(* Logix 5000 Rung export; software revision 16.04 *)

MODULES
   Local : vendor None type None code None
   PDPMV1_FLEX : vendor None type None code None
END_MODULES

TYPE PDPMV1_Status :   // Status data from the MVI56-PDPMV1 module
STRUCT
   Pattern : SINT[12];   // Module indentification code
   Input_Size : INT;   // Configured PROFIBUS input data size
   Output_Size : INT;   // Configured PROFIBUS output data size
   Reserved1 : INT;   // Not Used
   Reserved2 : INT;   // Not Used
   Reserved3 : INT;   // Not Used
   Input_Swap : SINT;   // Configured input swap byte option (1=swap bytes, 0= no swap)
   Output_Swap : SINT;   // Configured output swap byte option (1=swap bytes, 0= no swap)
   Module_Major_Ver : SINT;   // Module major firmware version
   Module_Minor_Ver : SINT;   // Module minor firmware version
   Fieldbus : PDPMV1_Fieldbus;   // PROFIBUS network status information
   Control : PDPMV1_StatusControl;   // Module information
   Profibus_CRC32 : DINT;   // CRC value related to the PROFIBUS configuration that was downloaded to the module
   Module_CRC32 : DINT;   // CRC value related to the module configuration that was downloaded to the module
   Module : PDPMV1_Module;   // General module status to monitor data, mailbox and alarm exchange between the processor and the module
   Backplane : PDPMV1_backplane;   // Backplane status information
   Other : PDPMV1_other_status;   // General mailbox and cfg error information
END_STRUCT
END_TYPE

TYPE PDPMV1_GetSlaveConfig_Out :   // GetSlaveConfig mailbox request
STRUCT
   SlaveAddress : INT;   // Destination of slave (1-125)
END_STRUCT
END_TYPE

TYPE PDPMV1_MSGUtil :   // Data structure for each MSG type that monitors if the message execution is sucessfull
STRUCT
   DNCounter : COUNTER;   // Incremented once the MSG done bit is set (PRE=100000)
   ERCounter : COUNTER;   // Incremented once the MSG ER bit is set (PRE=100000)
   LastError : INT;   // Last Error Code received
   Pending : BOOL;   // Indicates that the message is executing and the processor is waiting for its conclusion (DN or ER)
END_STRUCT
END_TYPE

TYPE PDPMV1_GetSlaveConfig_In :   // GetSlaveConfig mailbox response from a specific slave
STRUCT
   ByteCount : INT;   // Byte count data block
   SlaveAddress : INT;   // Destination of slave (1-125)
   ErrorCode : INT[1];   // If other than 0, refer to user manual for code information
   ReturnCode : INT;   // If other than 0, refer to user manual for code information
   FaultInformation : INT;   // If other than 0, refer to user manual for code information
   Identifier : SINT[245];   // Configuration from a specific connected PROFIBUS slave
END_STRUCT
END_TYPE

TYPE PDPMV1_StopSlave_Out :   // Mailbox request
STRUCT
   SlaveNumber : SINT[126];   // Slave number designation (1-125)
END_STRUCT
END_TYPE

TYPE PDPMV1_Control :   // This data structure contains the command bits to request mailbox, retrieve status and request reboot from the module
STRUCT
   AcyclicRead : BOOL;   // Request the module to send acyclic read message to slave
   AcyclicWrite : BOOL;   // Request the module to send acyclic write message to slave
   GetLiveList : BOOL;   // Request the Live List information from the module
   GetSlaveConfig : BOOL;   // Request configuration information from a slave
   GetSlaveDiagnostics : BOOL;   // Requests slave diagnostics from a slave
   GetStatus : BOOL;   // Request for status information from the module
   Reboot : BOOL;   // Request the module reboot
   SetClearMode : BOOL;   // Set the module to clear mode (outputs are disabled)
   SetOperateMode : BOOL;   // Set the module to operate mode (module only communicates through PROFIBUS)
   SetStopMode : BOOL;   // Set the module to stop mode (PROFIBUS communication is interrupted in stop mode)
   SetSlaveAddress : BOOL;   // Change the slave's PROFIBUS address (only if slave supports this feature)
   SetSlaveMode : BOOL;   // Set the slave mode to Synch, Freeze, Unsynch, Unfreeze
   StartSlaves : BOOL;   // Restarts PROFIBUS communication with one or more slaves after a "StopSlave" mailbox
   StopSlaves : BOOL;   // Stop PROFIBUS communication with one or more slaves
END_STRUCT
END_TYPE

TYPE PDPMV1_StartSlaves :   // StartSlaves mailbox allows the processor to restart communication to slaves that were previoulsy interrupted by StopSlaves
STRUCT
   Out : PDPMV1_StartSlaves_Out;   // Mailbox Request
   In : PDPMV1_StartSlaves_In;   // Mailbox Response
END_STRUCT
END_TYPE

TYPE PDPMV1_GetSlaveDiagnostics_In :   // GetSlaveDiagnostics mailbox response
STRUCT
   RequestType : SINT;   // Type of request. 0 to use module memory RAM or 1 for live PROFIBUS network.
   SlaveAddress : SINT;   // Destination of slave (1-125)
   ExtendedFaultInfo : INT;   // If other than 0, refer to user manual for code information
   FaultInformation : INT;   // If other than 0, refer to user manual for code information
   StationStatus1_2 : INT;   // Status of station types 1 and 2
   StationStatus3_4 : INT;   // Status of station types 3 and 4
   IdentNumber : INT;   // Unique ID assigned by the PROFIBUS User Organization
   ExtendedDiagnosticData : INT[200];   // Slave user-specific data. Refer to actual slave documentation for info
END_STRUCT
END_TYPE

TYPE PDPMV1_Alarm :   // DPV1 alarm data received by the module
STRUCT
   ByteCount : INT;   // Byte count data block
   SlotNumber : SINT;   // Used in the slave to address the desired data block. Range 0-254
   SlaveAddress : SINT;   // Destination of slave (1-125)
   AlarmSpecAck : SINT;   // Additional alarm information
   SeqNumber : SINT;   // Unique ID number of the alarm. Range 0-31.
   ExtDiag : SINT;   // Extended Diagnostic Flag (FFh - flag set and 00h - flag cleared).
   AlarmType : SINT;   // Identifies alarm type. Range is from 1 to 6, 32 to 126.
   FaultInformation : INT;   // If other than 0, refer to user manual for code information
   Data : SINT[500];   // Returned data [1...n] array with additional manf. spec alarm info.
END_STRUCT
END_TYPE

TYPE PDPMV1_Connection_Output :   // Connection input to be associated to the module
STRUCT
   Data : INT[69];   // Backplane output connection type - change the array size for your application
END_STRUCT
END_TYPE

TYPE PDPMV1_AcyclicRead_In :   // DPV1 acyclic read mailbox response
STRUCT
   ByteCount : INT;   // Byte count data block
   SlotNumber : SINT;   // Used in the slave to address the desired data block.
   SlaveAddress : SINT;   // Destination of slave (1-125)
   Length : SINT;   // Specifies the number of bytes of the data block to read
   Index : SINT;   // Index block
   ErrorDecode : SINT;   // If other than 0, refer to user manual for code information
   ErrorCode2 : SINT;   // If other than 0, refer to user manual for code information
   ErrorCode1 : SINT;   // If other than 0, refer to user manual for code information
   ExtendedFaultInfo : INT;   // If other than 0, refer to user manual for code information
   FaultInformation : INT;   // If other than 0, refer to user manual for code information
   Data : SINT[200];   // Returned data [1...n] array
END_STRUCT
END_TYPE

TYPE PDPMV1_PROFIBUS_IOSize :   // This type is used to store the module configuration input and output parameters
STRUCT
   InputDataSize : INT;   // Total PROFIBUS input word count configured through PCB.
   OutputDataSize : INT;   // Total PROFIBUS output word count configured through PCB.
END_STRUCT
END_TYPE

TYPE PDPMV1_AcyclicRead_Out :   // DPV1 acyclic read mailbox request
STRUCT
   SlotNumber : SINT;   // Used in the slave to address the desired data block.
   SlaveAddress : SINT;   // Destination of slave (1-125)
   DataSize : INT;   // Object data size
   Length : SINT;   // Specifies the number of bytes of the data block to read
   Index : SINT;   // Index block
END_STRUCT
END_TYPE

TYPE PDPMV1_UTIL :   // Contains registers used for ladder usage (these should not be updated by user application)
STRUCT
   CurrentAlarm : INT;   // New alarm index received from the module.
   CurrentMailbox : INT;   // New current mailbox index received from the module
   LastRead : INT;   // Last read block index received from the module
   ReadBlockIDOffset : INT;   // Read Block ID offset in Read Block
   LastWrite : INT;   // Last write block index received from the module
   BlockIndex : INT;   // Block index of each copy of PROFIBUS input and output blocks
   ReadBlockCount : INT;   // Number of read blocks transferred by the module to the processor
   WriteBlockCount : INT;   // Number of write blocks transferred by the processor to the module
   ReadBlockSize : INT;   // Input total size configured through RSLogix and reported by the module
   WriteBlockSize : INT;   // Output total size configured through RSLogix and reported by the module
   OutputWordsPerWriteBlock : INT;   // Word count reserved for PROFIBUS output data. All write blocks will use this amount except possibly last block.
   InputWordsPerReadBlock : INT;   // Word count reserved for PROFIBUS input data. All read blocks will use this amount except possibly last block.
   InputBytesPerReadBlock : INT;   // Byte count reserved for PROFIBUS input data. All read blocks will use this amount except possibly last block.
   OutputWordsInLastWriteBlock : INT;   // Word count with PROFIBUS output data in the last write block.
   InputWordsInLastReadBlock : INT;   // Word count with PROFIBUS input data in the last read block.
   InputBytesInLastReadBlock : INT;   // Byte count with PROFIBUS intput data in the last read block.
   MailboxInBuffer : INT[144];   // Mailbox response buffer received from the module. The content will be handled according to its mailbox ID
   MailboxOutBuffer : INT[144];   // Output mailbox buffer
   AlarmBuffer : INT[144];   // Buffer that stores the received alarm information
   StatusBuffer : INT[76];   // Buffer that stores the received status information
   MailboxIDOutLowByte : INT;   // Mailbox ID incremented for every mailbox request. Occupies the low byte of mailbox ID word register
   MailboxIDOut : INT;   // Final MailboxID for request mailbox. Corresponds to MailboxIDOutLowByte at low byte and "-20480" at high byte
   MailboxIDIn : INT;   // Received mailbox ID from the module - will match the corresponding request mailbox ID
   ByteSwapUtil : INT;   // Used for byte swap logic
   TempInt : INT;   // Used for integer formatting
   MSG : PDPMV1_MSGUtilTotal;   // Control Registers for MSG operation
END_STRUCT
END_TYPE

TYPE PDPMV1_AcyclicRead :   // DPV1 acyclic read mailbox data structure
STRUCT
   Out : PDPMV1_AcyclicRead_Out;   // mailbox request
   In : PDPMV1_AcyclicRead_In;   // mailbox response
END_STRUCT
END_TYPE

TYPE PDPMV1_SetSlaveMode :   // SetSlaveMode mailbox that allows the processor to change the slave mode to interrupt input or output data update
STRUCT
   Out : PDPMV1_SetSlaveMode_Out;   // Mailbox Request
   In : PDPMV1_SetSlaveMode_In;   // Mailbox Response
END_STRUCT
END_TYPE

TYPE PDPMV1_GetSlaveDiagnostics_Out :   // GetSlaveDiagnostics mailbox request
STRUCT
   RequestType : SINT;   // Type of request. 0 to use module memory RAM or 1 for live PROFIBUS network.
   SlaveAddress : SINT;   // Destination of slave (1-125)
END_STRUCT
END_TYPE

TYPE PDPMV1_Module :   // Status data
STRUCT
   Mod_scan_count : INT;   // Incremented every module scan loop
   Mod_output_update : INT;   // Incremented at every output scan
   Mod_input_update : INT;   // Incremented at every input scan
   Mod_out_MB : INT;   // Incremented at every output mailbox processing
   Mod_in_MB : INT;   // Incremented at every intput mailbox processing
   Mod_alarm_ind : INT;   // Incremented at every alarm indication
   Mod_alarm_con : INT;   // Incremented at every alarm confirmation
   Mod_acyclic_read : INT;   // Reserved
   Mod_acyclic_write : INT;   // Reserved
END_STRUCT
END_TYPE

TYPE PDPMV1_GetSlaveConfig :   // GetSlaveConfig mailobox to retrieve configuration data from specific PROFIBUS slaves
STRUCT
   Out : PDPMV1_GetSlaveConfig_Out;   // mailbox request
   In : PDPMV1_GetSlaveConfig_In;   // mailbox response
END_STRUCT
END_TYPE

TYPE PDPMV1_Connection_Input :   // Connection input to be associated to the module
STRUCT
   Data : INT[72];   // Backplane input connection type - change the array size for your application
END_STRUCT
END_TYPE

TYPE PDPMV1_GetSlaveDiagnostics :   // GetSlaveDiagnostics mailbox to retrieve diagnostic information from specific PROFIBUS slaves
STRUCT
   Out : PDPMV1_GetSlaveDiagnostics_Out;   // Mailbox request
   In : PDPMV1_GetSlaveDiagnostics_In;   // Mailbox response
END_STRUCT
END_TYPE

TYPE PDPMV1_StopSlave_In :   // Mailbox response
STRUCT
   AdditionalFaultinfo : INT;   // If other than 0, refer to user manual for code information
   FaultInformation : INT;   // If other than 0, refer to user manual for code information
   SlaveNumber : SINT[126];   // Slave number designation (1-125)
END_STRUCT
END_TYPE

TYPE PDPMV1_StartSlaves_In :   // Mailbox Response
STRUCT
   AdditionalFaultInfo : INT;   // If other than 0, refer to user manual for code information
   FaultInformation : INT;   // If other than 0, refer to user manual for code information
   SlaveNumber : SINT[126];   // Slave number designation (1-125)
END_STRUCT
END_TYPE

TYPE PDPMV1_GetLiveList :   // GetLiveList mailbox to retrieve the live list information from PROFIBUS network, informing the slaves that are communicating
STRUCT
   ReturnCode : SINT;   // Returned code about the nodes on the network
   FaultInfo : SINT;   // If other than 0, refer to user manual for code information
   Station : SINT[127];   // Station type contents.
END_STRUCT
END_TYPE

TYPE PDPMV1_ModuleDefinition :   // Main module definition
STRUCT
   PROFIBUSData : PDPMV1_Data;   // PROFIBUS data transferred between the processor and the PROFIBUS network
   Config : PDPMV1_Configuration;   // Module configuration information (backplane block sizes and PROFIBUS data sizes)
   Command : PDPMV1_Control;   // Command bits for special tasks and mailbox requests
   Mailbox : PDPMV1_Mailbox;   // Mailbox tags for optional applications
   Status : PDPMV1_Status;   // Module status information
   Util : PDPMV1_UTIL;   // Internal tags used for ladder logic processing. User applications should not overwrite any Util tags
END_STRUCT
END_TYPE

TYPE PDPMV1_Mailbox :   // Stores all mailbox request and response registers
STRUCT
   AcyclicRead : PDPMV1_AcyclicRead;   // This encapsulates a DPV1 Class 1 acyclic read request.
   AcyclicWrite : PDPMV1_AcyclicWrite;   // This encapsulates a DPV1 Class 1 acyclic write request.
   Alarm : PDPMV1_Alarm;   // This indicates to the application that a DPV1 slave has transferred an Alarm message to the master.
   GetLiveList : PDPMV1_GetLiveList;   // This command returns 127 bytes of information about the nodes on the network.
   GetSlaveConfig : PDPMV1_GetSlaveConfig;   // This command reads the actual configuration (identifier bytes) of a specified slave.
   GetSlaveDiagnostics : PDPMV1_GetSlaveDiagnostics;   // This command reads diagnostic data from a specified slave.
   SetSlaveAddress : PDPMV1_SetSlaveAddress;   // This command makes it possible to set the node address of a specified slave, if the slave supports this feature.
   SetSlaveMode : PDPMV1_SetSlaveMode;   // This control command is transmitted as multicast commands.
   StartSlaves : PDPMV1_StartSlaves;   // This mailbox message starts a selection of slaves that was previously removed from the processing cycle by means of the mailbox
   StopSlaves : PDPMV1_StopSlave;   // This mailbox message stops a selection of slaves from the processing cycle.
END_STRUCT
END_TYPE

TYPE PDPMV1_SetSlaveMode_In :   // Mailbox response
STRUCT
   GroupSelect : SINT;   // Range 01h to FFh (Bit Coded). This parameter determines which group to address. Refer to the user manual for examples
   SlaveAddress : SINT;   // Range 1 to 125; 127 (Multicast address).
   ControlCommand : PDPMV1_ControlCommand;   // This parameter specifies the command to send (Unsync/Sync and Unfreeze/Freeze).
   ExtendedFaultInfo : INT;   // If other than 0, refer to user manual for code information
   FaultInformation : INT;   // If other than 0, refer to user manual for code information
END_STRUCT
END_TYPE

TYPE PDPMV1_AcyclicWrite_In :   // DPV1 acyclic write mailbox response
STRUCT
   ByteCount : INT;   // Byte count data block
   SlotNumber : SINT;   // Used in the slave to address the desired data block.
   SlaveAddress : SINT;   // Destination of slave (1-125)
   Length : SINT;   // Specifies the number of bytes of the data block to read
   Index : SINT;   // Index block
   ErrorDecode : SINT;   // If other than 0, refer to user manual for code information
   ErrorCode2 : SINT;   // If other than 0, refer to user manual for code information
   ErrorCode1 : SINT;   // If other than 0, refer to user manual for code information
   ExtendedFaultInfo : INT;   // If other than 0, refer to user manual for code information
   FaultInformation : INT;   // If other than 0, refer to user manual for code information
   Data : SINT[200];   // Returned data [1...n] array
END_STRUCT
END_TYPE

TYPE PDPMV1_SetSlaveAddress_In :   // Mailbox response
STRUCT
   ByteCount : INT;   // Byte count data block
   NewSlaveAddress : SINT;   // Range 1 to 125, specifies the new address of the slave.
   CurrentSlaveAddress : SINT;   // Range 1 to 125, specifies the current address of the slave.
   SlaveIdentNumber : INT;   // Ident number for the slave, which address should be altered.
   No_add_Chg : INT;   // This parameter specifies whether it is allowed to change the slave address again
   ErrorCode1_2 : INT;   // If other than 0, refer to user manual for code information
   ErrorCode3_4 : INT;   // If other than 0, refer to user manual for code information
   ReturnCode : INT;   // If other than 0, refer to user manual for code information
   FaultInformation : INT;   // If other than 0, refer to user manual for code information
   MessageDataByte : SINT[400];   // Message data byte array for user-specific data
END_STRUCT
END_TYPE

TYPE PDPMV1_StatusControl :   // Module general information
STRUCT
   serial_number : SINT[4];   // Module serial number
   version_MSB : SINT;   // Module version number (most significant byte)
   version_LSB : SINT;   // Module version number (least significant byte)
   mod_status_MSB : SINT;   // Module status (most significant byte)
   mod_status_LSB : SINT;   // Module status (least significant byte)
END_STRUCT
END_TYPE

TYPE PDPMV1_ControlCommand :   // Option bits for SetSlaveMode mailbox
STRUCT
   Reserved1 : BOOL;   // Reserved
   Reserved2 : BOOL;   // Reserved
   Unfreeze_Input : BOOL;   // Freeze mode is concluded when initiated
   Freeze_Input : BOOL;   // Causes the addressed slave to assume freeze mode.
   Unsynchronize_Output : BOOL;   // Unsynchronized output data
   Synchronize_Output : BOOL;   // Synchronized output data
   Reserved3 : BOOL[32];   // Reserved
END_STRUCT
END_TYPE

TYPE PDPMV1_SetSlaveMode_Out :   // Mailbox Request
STRUCT
   GroupSelect : SINT;   // Range 01h to FFh (Bit Coded). This parameter determines which group to address. Refer to the user manual for examples
   SlaveAddress : SINT;   // Range 1 to 125; 127 (Multicast address).
   ControlCommand : PDPMV1_ControlCommand;   // This parameter specifies the command to send (Unsync/Sync and Unfreeze/Freeze).
END_STRUCT
END_TYPE

TYPE PDPMV1_Backplane_IOSize :   // This type is used to store the module configuration input and output parameters
STRUCT
   ReadBlockSize : INT;   // Total read (input) block size in words set for 1756-MODULE profile through RSLogix (from 12 through 250 words)
   WriteBlockSize : INT;   // Total write (output) block size in words set for 1756-MODULE profile through RSLogix (from 5 through 248 words)
END_STRUCT
END_TYPE

TYPE PDPMV1_StartSlaves_Out :   // Mailbox Request
STRUCT
   SlaveNumber : SINT[126];   // Slave number designation (1-125)
END_STRUCT
END_TYPE

TYPE PDPMV1_SetSlaveAddress :   // SetSlaveAddress mailbox that allows the module to dynamically change a PRIDUBUS address (only for slaves that supports it)
STRUCT
   Out : PDPMV1_SetSlaveAddress_Out;   // Mailbox request
   In : PDPMV1_SetSlaveAddress_In;   // Mailbox response
END_STRUCT
END_TYPE

TYPE PDPMV1_MSGUtilTotal :   // Stores all registers that are used to monitor MSG execution.
STRUCT
   MailboxRequest : PDPMV1_MSGUtil;   // Registers for monitoring of request mailbox MSG instructions
   MailboxResponse : PDPMV1_MSGUtil;   // Registers for monitoring of response mailbox MSG instructions
   GetStatus : PDPMV1_MSGUtil;   // Registers for monitoring of get status MSG instructions
   GetAlarm : PDPMV1_MSGUtil;   // Registers for monitoring of rget alarm MSG instructions
END_STRUCT
END_TYPE

TYPE PDPMV1_AcyclicWrite :   // DPV1 acyclic write mailbox data structure
STRUCT
   Out : PDPMV1_AcyclicWrite_Out;   // Mailbox request
   In : PDPMV1_AcyclicWrite_In;   // Mailbox response
END_STRUCT
END_TYPE

TYPE PDPMV1_StopSlave :   // StopSlaves mailbox allows the processor to interrupt communication to specific PROFIBUS slaves
STRUCT
   Out : PDPMV1_StopSlave_Out;   // Mailbox Request
   In : PDPMV1_StopSlave_In;   // Mailbox Response
END_STRUCT
END_TYPE

TYPE PDPMV1_SetSlaveAddress_Out :   // Mailbox request
STRUCT
   ByteCount : INT;   // Byte count data block
   NewSlaveAddress : SINT;   // Range 1 to 125, specifies the new address of the slave.
   CurrentSlaveAddress : SINT;   // Range 1 to 125, specifies the current address of the slave.
   SlaveIdentNumber : INT;   // Ident number for the slave, which address should be altered.
   No_add_Chg : INT;   // This parameter specifies whether it is allowed to change the slave address again
   MessageDataByte : SINT[400];   // Message data byte array for user-specific data
END_STRUCT
END_TYPE

TYPE PDPMV1_Data :   // PROFIBUS data transferred between the processor and and the PROFIBUS slaves
STRUCT
   Input : SINT[1536];   // Input PROFIBUS data (from module to processor)
   Output : SINT[1536];   // Output PROFIBUS data (from processor to module)
END_STRUCT
END_TYPE

TYPE PDPMV1_backplane :   // Stores variables used by sample ladder logic for handshaking purposes.
STRUCT
   Read : INT;   // Backplane read statistics
   Write : INT;   // Backplane write statistics
   Error : INT;   // Backplane error statistics
END_STRUCT
END_TYPE

TYPE PDPMV1_other_status :
STRUCT
   Cfg_file_error : INT;   // Bit0 = PDPMV1.CFG, Bit 1 = WATTCP.CFG, Bit 2 = PDPMV1.DDB, Bit3=PDPMV1.XML
   Reserved0 : INT;   // Not Used
   Reserved1 : INT;   // Not Used
   Reserved2 : INT;   // Not Used
   Reserved3 : INT;   // Not Used
   Reserved4 : INT;   // Not Used
   Reserved5 : INT;   // Not Used
   Reserved6 : INT;   // Not Used
   Reserved7 : INT;   // Not Used
   Reserved8 : INT;   // Not Used
   Reserved9 : INT;   // Not Used
   Reserved10 : INT;   // Not Used
   Reserved11 : INT;   // Not Used
   Reserved12 : INT;   // Not Used
   In_MB_queue : INT;   // Number of messages in the input mailbox queue
   Out_MB_queue : INT;   // Number of messages in the output mailbox queue
   Alarm_MB_queue : INT;   // Number of messages in the alarm mailbox queue
END_STRUCT
END_TYPE

TYPE PDPMV1_Fieldbus :
STRUCT
   FB_Slave_Cfg_List : SINT[16];   // Bitmap structure containing PROFIBUS slave configuration (bit x = 1 means slave x is configured)
   FB_Slave_Data_xfer : SINT[16];   // Bitmap structure containing PROFIBUS slave data exchange status (bit x = 1 means slave x is transferring data to the module)
   FB_Slave_Diag : SINT[16];   // Bitmap structure containing PROFIBUS slave diagnostic info (bit x = 1 means slave x is reporting diagnostics)
   FB_Pad_Byte : SINT;   // Reserved
   FB_op_state : SINT;   // Operation state ( 00 = offline, 40 = stop, 80 = clear, C0= operate)
   FB_ident_MSB : SINT;   // Master identification code (most significant byte)
   FB_ident_LSB : SINT;   // Master identification code (least significant byte)
END_STRUCT
END_TYPE

TYPE PDPMV1_Configuration :   // Stores current module configuration read from the module. The module cannot be configured from ladder.
STRUCT
   Backplane : PDPMV1_Backplane_IOSize;   // This tag will contain the input and output backplane block sizes configured by the user for the module through RSLogix
   PROFIBUS : PDPMV1_PROFIBUS_IOSize;   // This tag will contain the input and output PROFIBUS sizes configured by the user for the module through PCB
   PROFIBUS_CRC : DINT;   // Contains the CRC value (32-bits) associated to the module configuration file
   Module_CRC : DINT;   // Contains the CRC value (32-bits) associated to the PROFIBUSconfiguration file
END_STRUCT
END_TYPE

TYPE PDPMV1_AcyclicWrite_Out :   // DPV1 acyclic write mailbox request
STRUCT
   SlotNumber : SINT;   // Used in the slave to address the desired data block.
   SlaveAddress : SINT;   // Destination of slave (1-125)
   DataSize : INT;   // Object data size
   Length : SINT;   // Specifies the number of bytes of the data block to read
   Index : SINT;   // Index block
   Data : SINT[200];   // Data that should be written [1...n]
END_STRUCT
END_TYPE

ADD_ON_INSTRUCTION AOI56PDPMV1_FLEX   (* revision 1.5, vendor ProSoft Technology Inc., ExecutePrescan *)
// Add-On for the MVI56-PDPMV1 (Flexible I/O) module.
// Revision note:
// v1.5 - Commands that require messaging can now be accessed more than once after power up or mode change.
VAR_IN_OUT
   Connection_Input : PDPMV1_Connection_Input; {required}
   Connection_Output : PDPMV1_Connection_Output; {required}
   MVI56PDPMV1 : PDPMV1_ModuleDefinition; {required}
   AcyclicRead_MSG : MESSAGE; {required}   // Message tag for Acyclic Read mailbox request
   AcyclicWrite_MSG : MESSAGE; {required}   // Message tag for Acyclic Write mailbox request
   GetAlarm_MSG : MESSAGE; {required}   // Message tag for Get Alarm mailbox request
   GetMailbox_MSG : MESSAGE; {required}   // Message tag to retrieve mailbox response
   GetStatus_MSG : MESSAGE; {required}   // Message tag to retrieve module status
   GetLiveList_MSG : MESSAGE; {required}   // Message tag for Get Live List mailbox request
   GetSlaveCfg_MSG : MESSAGE; {required}   // Message tag for Get Slave Configuration mailbox request
   GetSlaveDiagnostics_MSG : MESSAGE; {required}   // Message tag for Get Slave Diagnostics mailbox request
   SetClearMode_MSG : MESSAGE; {required}   // Message tag for Set Clear Mode mailbox request
   SetOperateMode_MSG : MESSAGE; {required}   // Message tag for Set Operate Mode mailbox request
   SetSlaveAddress_MSG : MESSAGE; {required}   // Message tag for Set Slave Address mailbox request
   SetSlaveMode_MSG : MESSAGE; {required}   // Message tag for Set Slave Mode mailbox
   SetStopMode_MSG : MESSAGE; {required}   // Message tag for Set Stop mode mailbox request
   StartSlaves_MSG : MESSAGE; {required}   // Message tag for Start Slaves mailbox request
   StopSlaves_MSG : MESSAGE; {required}   // Message tag for Stop Slaves mailbox request
END_VAR
VAR
   MJFAULTS : DINT[12];
END_VAR

ROUTINE Logic   (* ladder *)
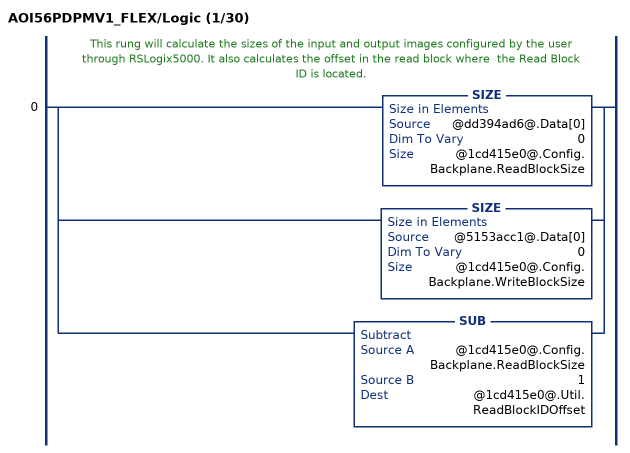
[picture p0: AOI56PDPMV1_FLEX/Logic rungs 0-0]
   // This rung will calculate the sizes of the input and output images configured by the user through RSLogix5000. It also calculates the offset in the read block where  the Read Block ID is located.
   0: [SIZE(@dd394ad6@.Data[0],0,@1cd415e0@.Config.Backplane.ReadBlockSize) ,SIZE(@5153acc1@.Data[0],0,@1cd415e0@.Config.Backplane.WriteBlockSize) ,SUB(@1cd415e0@.Config.Backplane.ReadBlockSize,1,@1cd415e0@.Util.ReadBlockIDOffset) ];
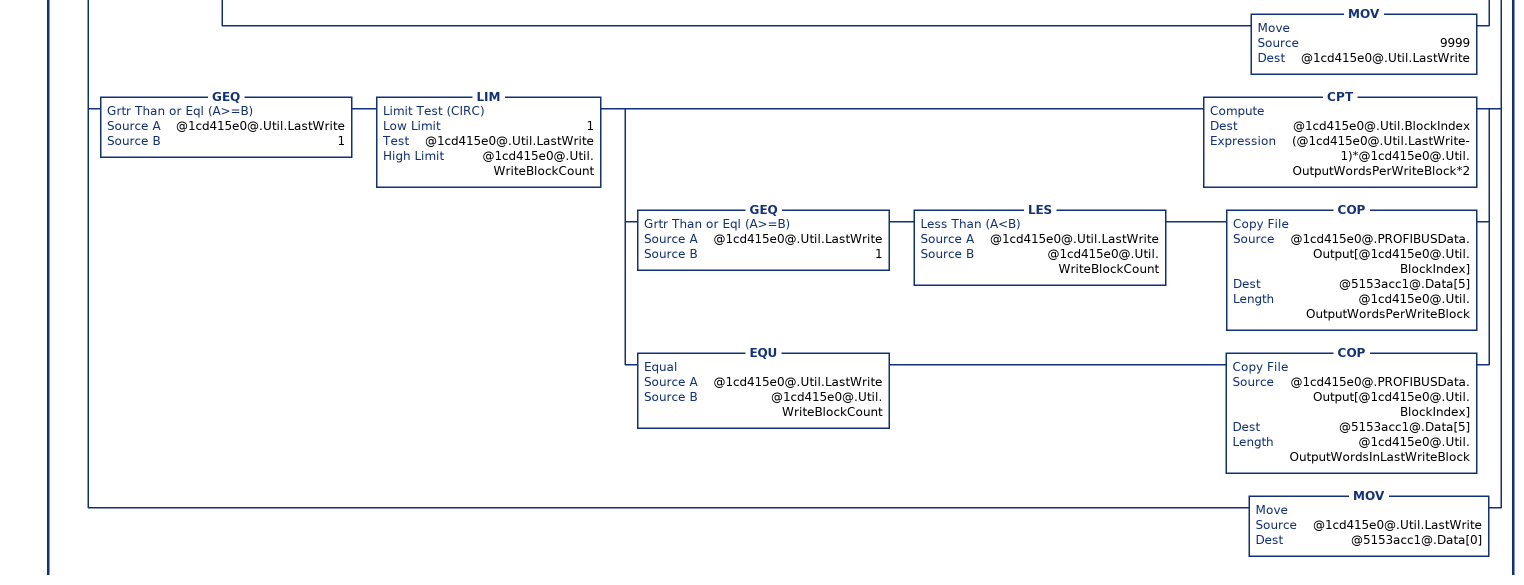
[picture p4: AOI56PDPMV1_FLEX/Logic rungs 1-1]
   // The new received read block ID is copied to the MVI56PDPMV1.Util.LastRead controller tag to guarantee that this logic will be performed one time only for each new bloc.
   1: NEQ(@dd394ad6@.Data[@1cd415e0@.Util.ReadBlockIDOffset],@1cd415e0@.Util.LastRead)[MOV(@dd394ad6@.Data[@1cd415e0@.Util.ReadBlockIDOffset],@1cd415e0@.Util.LastRead) ,EQU(@dd394ad6@.Data[0],9990) EQU(@1cd415e0@.Util.LastRead,9990) [MOV(@dd394ad6@.Data[1],@1cd415e0@.Util.ReadBlockSize) ,MOV(@dd394ad6@.Data[2],@1cd415e0@.Util.WriteBlockSize) ,MOV(@dd394ad6@.Data[3],@1cd415e0@.Config.PROFIBUS.InputDataSize) ,MOV(@dd394ad6@.Data[4],@1cd415e0@.Config.PROFIBUS.OutputDataSize) ,MOV(@dd394ad6@.Data[5],@1cd415e0@.Util.ReadBlockCount) ,MOV(@dd394ad6@.Data[6],@1cd415e0@.Util.WriteBlockCount) ,MOV(@dd394ad6@.Data[7],@1cd415e0@.Util.InputWordsPerReadBlock) ,MUL(@1cd415e0@.Util.InputWordsPerReadBlock,2,@1cd415e0@.Util.InputBytesPerReadBlock) ,MOV(@dd394ad6@.Data[8],@1cd415e0@.Util.OutputWordsPerWriteBlock) ,MOV(@dd394ad6@.Data[9],@1cd415e0@.Util.InputWordsInLastReadBlock) ,MUL(@1cd415e0@.Util.InputWordsInLastReadBlock,2,@1cd415e0@.Util.InputBytesInLastReadBlock) ,MOV(@dd394ad6@.Data[10],@1cd415e0@.Util.OutputWordsInLastWriteBlock) ,MOV(0,@1cd415e0@.Util.CurrentAlarm) ,MOV(0,@1cd415e0@.Util.CurrentMailbox) ,OTU(@1cd415e0@.Util.MSG.MailboxRequest.Pending) ] ,GEQ(@1cd415e0@.Util.LastRead,0) LIM(0,@1cd415e0@.Util.LastRead,@1cd415e0@.Util.ReadBlockCount) [COP(@dd394ad6@.Data[1],@1cd415e0@.Config.PROFIBUS_CRC,2) ,COP(@dd394ad6@.Data[5],@1cd415e0@.Util.CurrentMailbox,1) ,COP(@dd394ad6@.Data[6],@1cd415e0@.Util.CurrentAlarm,1) ,GRT(@1cd415e0@.Util.LastRead,0) CPT(@1cd415e0@.Util.BlockIndex,(@1cd415e0@.Util.LastRead-1)*@1cd415e0@.Util.InputWordsPerReadBlock*2) ,EQU(@1cd415e0@.Util.LastRead,0) MOV(0,@1cd415e0@.Util.BlockIndex) ,GEQ(@1cd415e0@.Util.LastRead,0) LES(@1cd415e0@.Util.LastRead,@1cd415e0@.Util.ReadBlockCount) COP(@dd394ad6@.Data[7],@1cd415e0@.PROFIBUSData.Input[@1cd415e0@.Util.BlockIndex],@1cd415e0@.Util.InputBytesPerReadBlock) ,EQU(@1cd415e0@.Util.LastRead,@1cd415e0@.Util.ReadBlockCount) COP(@dd394ad6@.Data[7],@1cd415e0@.PROFIBUSData.Input[@1cd415e0@.Util.BlockIndex],@1cd415e0@.Util.InputBytesInLastReadBlock) ] ,EQU(@1cd415e0@.Util.LastRead,-1) [COP(@dd394ad6@.Data[1],@1cd415e0@.Config.PROFIBUS_CRC,2) ,COP(@dd394ad6@.Data[5],@1cd415e0@.Util.CurrentMailbox,1) ,COP(@dd394ad6@.Data[6],@1cd415e0@.Util.CurrentAlarm,1) ] ,MOV(@dd394ad6@.Data[0],@1cd415e0@.Util.LastWrite) ,COP(@1cd415e0@.Config.PROFIBUS_CRC,@5153acc1@.Data[1],4) ,XIC(@1cd415e0@.Command.Reboot) [OTU(@1cd415e0@.Command.Reboot) ,MOV(9999,@1cd415e0@.Util.LastWrite) ] ,GEQ(@1cd415e0@.Util.LastWrite,1) LIM(1,@1cd415e0@.Util.LastWrite,@1cd415e0@.Util.WriteBlockCount) [CPT(@1cd415e0@.Util.BlockIndex,(@1cd415e0@.Util.LastWrite-1)*@1cd415e0@.Util.OutputWordsPerWriteBlock*2) ,GEQ(@1cd415e0@.Util.LastWrite,1) LES(@1cd415e0@.Util.LastWrite,@1cd415e0@.Util.WriteBlockCount) COP(@1cd415e0@.PROFIBUSData.Output[@1cd415e0@.Util.BlockIndex],@5153acc1@.Data[5],@1cd415e0@.Util.OutputWordsPerWriteBlock) ,EQU(@1cd415e0@.Util.LastWrite,@1cd415e0@.Util.WriteBlockCount) COP(@1cd415e0@.PROFIBUSData.Output[@1cd415e0@.Util.BlockIndex],@5153acc1@.Data[5],@1cd415e0@.Util.OutputWordsInLastWriteBlock) ] ,MOV(@1cd415e0@.Util.LastWrite,@5153acc1@.Data[0]) ];
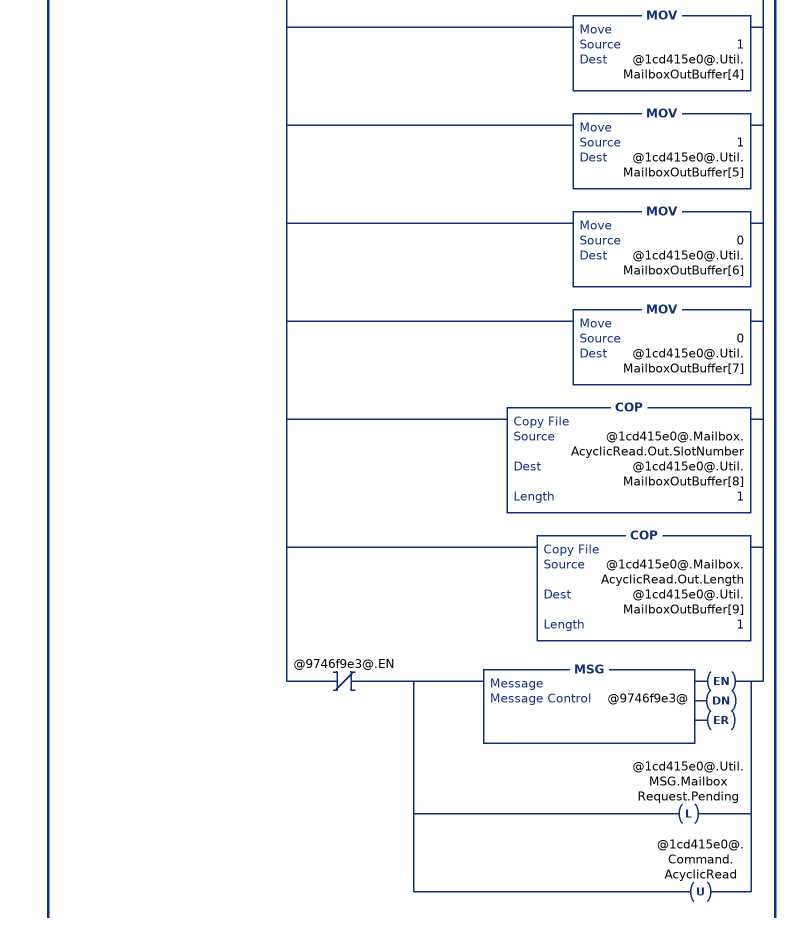
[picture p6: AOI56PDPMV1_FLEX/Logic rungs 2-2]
   // Acyclic Read mailbox request.
   // Allows the acyclic read of DPV1 information from a specific PROFIBUS slave.
   // This rung initially creates a new mailbox ID by incrementing the last sent mailbox ID by a value of 1.  The mailbox ID is composed of the low byte containing the new mailbox ID and the high byte containing the decimal value of "-20480" (indicating the mailbox from the backplane).
   // This rung will update the MVI56PDPMV1.Util.MailboxOutBuffer according to the specific mailbox request and then execute the MSG instruction.  The MVI56PDPMV1.Util.MSG.MailboxRequest.Pending will be latched until the MSG operation is concluded to prevent other mailbox requests to be performed during that time. If the MSG operation is successfull then the MVI56PDPMV1.Util.MSG.MailboxRequest.DNCounter tag is incremented and the DN bit is cleared. If the MSG is not sucessfull then the MVI56PDPMV1.Util.MSG.MailboxRequest.ERCounter is incremented and the ER bit is cleared. A minimum of 100ms time should be kept between two consecutive requests for better performance, otherwise a MSG error might be returned.
   2: XIC(@1cd415e0@.Command.AcyclicRead)XIO(@1cd415e0@.Util.MSG.MailboxRequest.Pending)[[ADD(1,@1cd415e0@.Util.MailboxIDOutLowByte,@1cd415e0@.Util.MailboxIDOutLowByte) ,GEQ(@1cd415e0@.Util.MailboxIDOutLowByte,256) MOV(1,@1cd415e0@.Util.MailboxIDOutLowByte) ,ADD(@1cd415e0@.Util.MailboxIDOutLowByte,-20480,@1cd415e0@.Util.MailboxIDOut) ] ,MOV(@1cd415e0@.Util.MailboxIDOut,@1cd415e0@.Util.MailboxOutBuffer[0]) ,MOV(16386,@1cd415e0@.Util.MailboxOutBuffer[1]) ,MOV(32,@1cd415e0@.Util.MailboxOutBuffer[2]) ,COP(@1cd415e0@.Mailbox.AcyclicRead.Out.DataSize,@1cd415e0@.Mailbox.AcyclicRead.Out.Length,1) ,MOV(0,@1cd415e0@.Util.MailboxOutBuffer[3]) ,MOV(1,@1cd415e0@.Util.MailboxOutBuffer[4]) ,MOV(1,@1cd415e0@.Util.MailboxOutBuffer[5]) ,MOV(0,@1cd415e0@.Util.MailboxOutBuffer[6]) ,MOV(0,@1cd415e0@.Util.MailboxOutBuffer[7]) ,COP(@1cd415e0@.Mailbox.AcyclicRead.Out.SlotNumber,@1cd415e0@.Util.MailboxOutBuffer[8],1) ,COP(@1cd415e0@.Mailbox.AcyclicRead.Out.Length,@1cd415e0@.Util.MailboxOutBuffer[9],1) ,XIO(@9746f9e3@.EN) [MSG(@9746f9e3@) ,OTL(@1cd415e0@.Util.MSG.MailboxRequest.Pending) ,OTU(@1cd415e0@.Command.AcyclicRead) ] ];
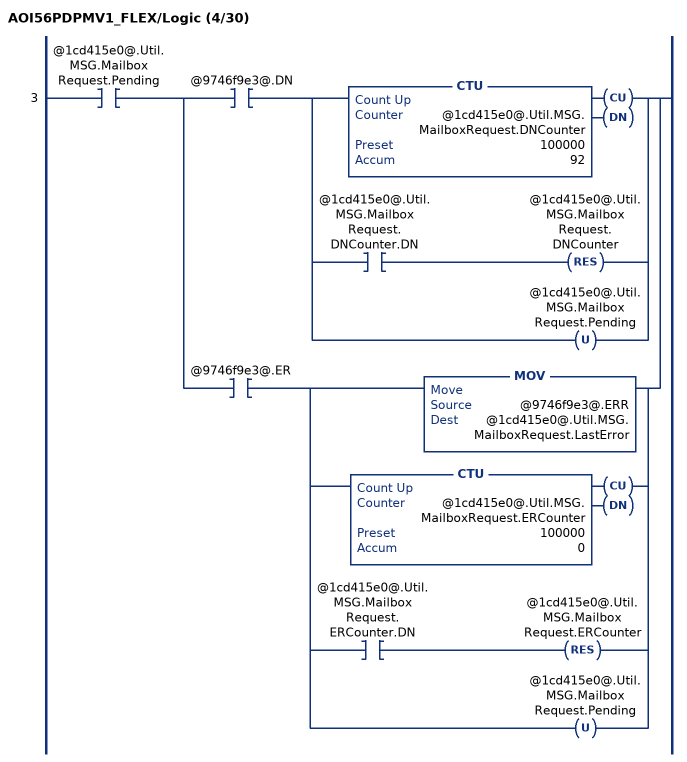
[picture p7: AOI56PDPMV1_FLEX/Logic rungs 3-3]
   3: XIC(@1cd415e0@.Util.MSG.MailboxRequest.Pending)[XIC(@9746f9e3@.DN) [CTU(@1cd415e0@.Util.MSG.MailboxRequest.DNCounter,100000,92) ,XIC(@1cd415e0@.Util.MSG.MailboxRequest.DNCounter.DN) RES(@1cd415e0@.Util.MSG.MailboxRequest.DNCounter) ,OTU(@1cd415e0@.Util.MSG.MailboxRequest.Pending) ] ,XIC(@9746f9e3@.ER) [MOV(@9746f9e3@.ERR,@1cd415e0@.Util.MSG.MailboxRequest.LastError) ,CTU(@1cd415e0@.Util.MSG.MailboxRequest.ERCounter,100000,0) ,XIC(@1cd415e0@.Util.MSG.MailboxRequest.ERCounter.DN) RES(@1cd415e0@.Util.MSG.MailboxRequest.ERCounter) ,OTU(@1cd415e0@.Util.MSG.MailboxRequest.Pending) ] ];
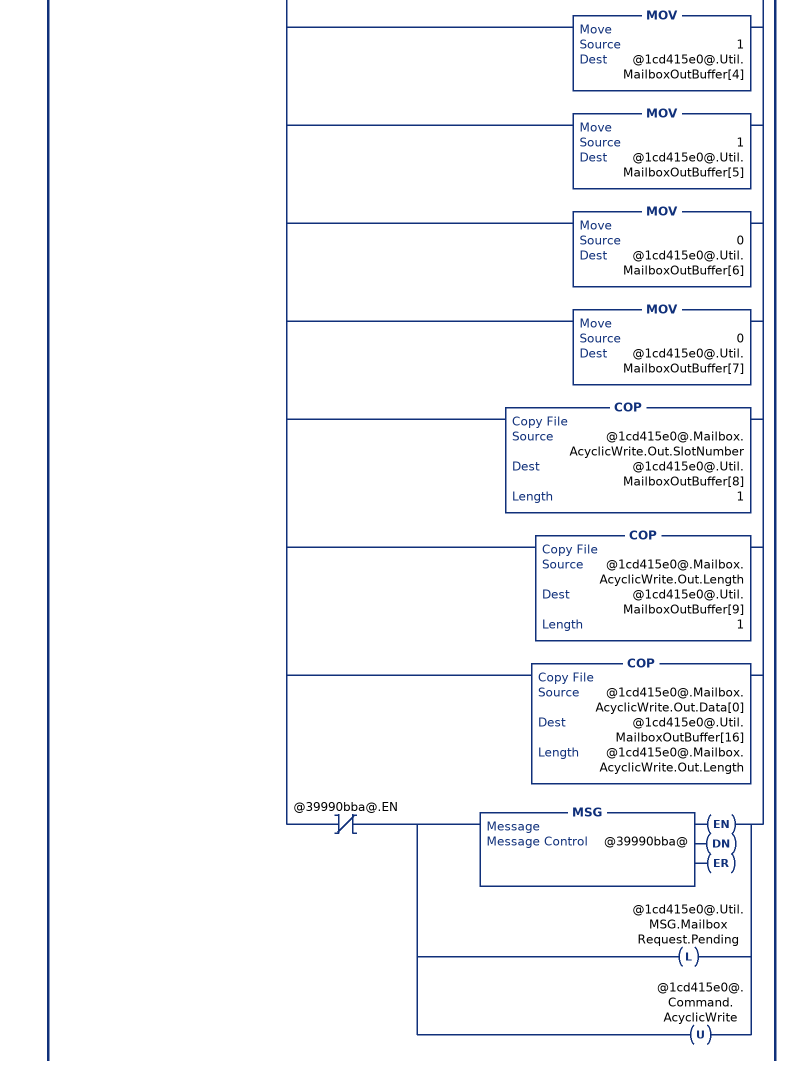
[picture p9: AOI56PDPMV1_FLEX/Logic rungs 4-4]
   // Acyclic Write mailbox request.
   // Allows the acyclic write of DPV1 information to a specific PROFIBUS slave.
   // This rung initially creates a new mailbox ID by incrementing the last sent mailbox ID by a value of 1.  The mailbox ID is composed of the low byte containing the new mailbox ID and the high byte containing the decimal value of "-20480" (indicating the mailbox from the backplane).
   // This rung will update the MVI56PDPMV1.Util.MailboxOutBuffer according to the specific mailbox request and then execute the MSG instruction.  The MVI56PDPMV1.Util.MSG.MailboxRequest.Pending will be latched until the MSG operation is concluded to prevent other mailbox requests to be performed during that time. If the MSG operation is successfull then the MVI56PDPMV1.Util.MSG.MailboxRequest.DNCounter tag is incremented and the DN bit is cleared. If the MSG is not sucessfull then the MVI56PDPMV1.Util.MSG.MailboxRequest.ERCounter is incremented and the ER bit is cleared. A minimum of 100ms time should be kept between two consecutive requests for better performance, otherwise a MSG error might be returned.
   4: XIC(@1cd415e0@.Command.AcyclicWrite)XIO(@1cd415e0@.Util.MSG.MailboxRequest.Pending)[[ADD(1,@1cd415e0@.Util.MailboxIDOutLowByte,@1cd415e0@.Util.MailboxIDOutLowByte) ,GEQ(@1cd415e0@.Util.MailboxIDOutLowByte,256) MOV(1,@1cd415e0@.Util.MailboxIDOutLowByte) ,ADD(@1cd415e0@.Util.MailboxIDOutLowByte,-20480,@1cd415e0@.Util.MailboxIDOut) ] ,MOV(@1cd415e0@.Util.MailboxIDOut,@1cd415e0@.Util.MailboxOutBuffer[0]) ,MOV(16386,@1cd415e0@.Util.MailboxOutBuffer[1]) ,MOV(33,@1cd415e0@.Util.MailboxOutBuffer[2]) ,COP(@1cd415e0@.Mailbox.AcyclicWrite.Out.DataSize,@1cd415e0@.Mailbox.AcyclicWrite.Out.Length,1) ,MOV(@1cd415e0@.Mailbox.AcyclicWrite.Out.DataSize,@1cd415e0@.Util.MailboxOutBuffer[3]) ,MOV(1,@1cd415e0@.Util.MailboxOutBuffer[4]) ,MOV(1,@1cd415e0@.Util.MailboxOutBuffer[5]) ,MOV(0,@1cd415e0@.Util.MailboxOutBuffer[6]) ,MOV(0,@1cd415e0@.Util.MailboxOutBuffer[7]) ,COP(@1cd415e0@.Mailbox.AcyclicWrite.Out.SlotNumber,@1cd415e0@.Util.MailboxOutBuffer[8],1) ,COP(@1cd415e0@.Mailbox.AcyclicWrite.Out.Length,@1cd415e0@.Util.MailboxOutBuffer[9],1) ,COP(@1cd415e0@.Mailbox.AcyclicWrite.Out.Data[0],@1cd415e0@.Util.MailboxOutBuffer[16],@1cd415e0@.Mailbox.AcyclicWrite.Out.Length) ,XIO(@39990bba@.EN) [MSG(@39990bba@) ,OTL(@1cd415e0@.Util.MSG.MailboxRequest.Pending) ,OTU(@1cd415e0@.Command.AcyclicWrite) ] ];
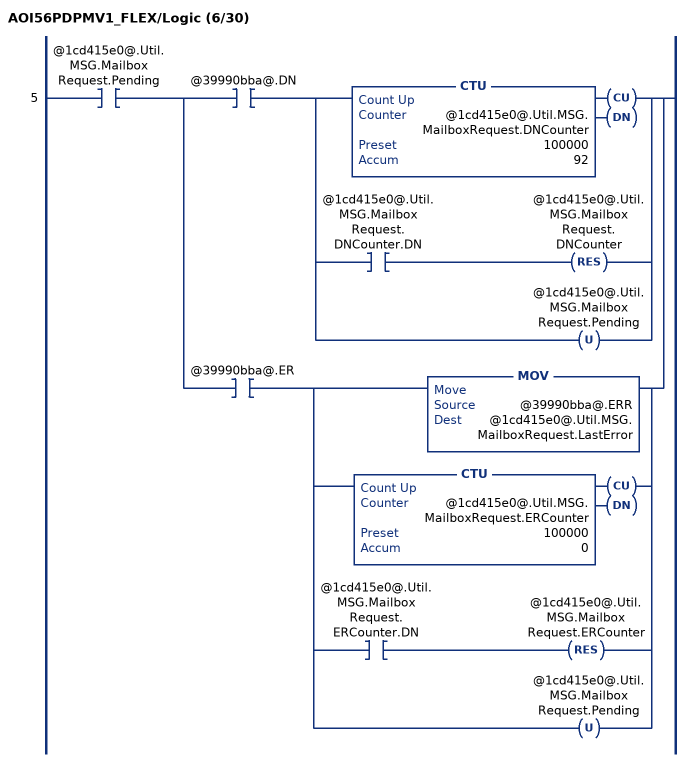
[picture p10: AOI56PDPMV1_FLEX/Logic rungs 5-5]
   5: XIC(@1cd415e0@.Util.MSG.MailboxRequest.Pending)[XIC(@39990bba@.DN) [CTU(@1cd415e0@.Util.MSG.MailboxRequest.DNCounter,100000,92) ,XIC(@1cd415e0@.Util.MSG.MailboxRequest.DNCounter.DN) RES(@1cd415e0@.Util.MSG.MailboxRequest.DNCounter) ,OTU(@1cd415e0@.Util.MSG.MailboxRequest.Pending) ] ,XIC(@39990bba@.ER) [MOV(@39990bba@.ERR,@1cd415e0@.Util.MSG.MailboxRequest.LastError) ,CTU(@1cd415e0@.Util.MSG.MailboxRequest.ERCounter,100000,0) ,XIC(@1cd415e0@.Util.MSG.MailboxRequest.ERCounter.DN) RES(@1cd415e0@.Util.MSG.MailboxRequest.ERCounter) ,OTU(@1cd415e0@.Util.MSG.MailboxRequest.Pending) ] ];
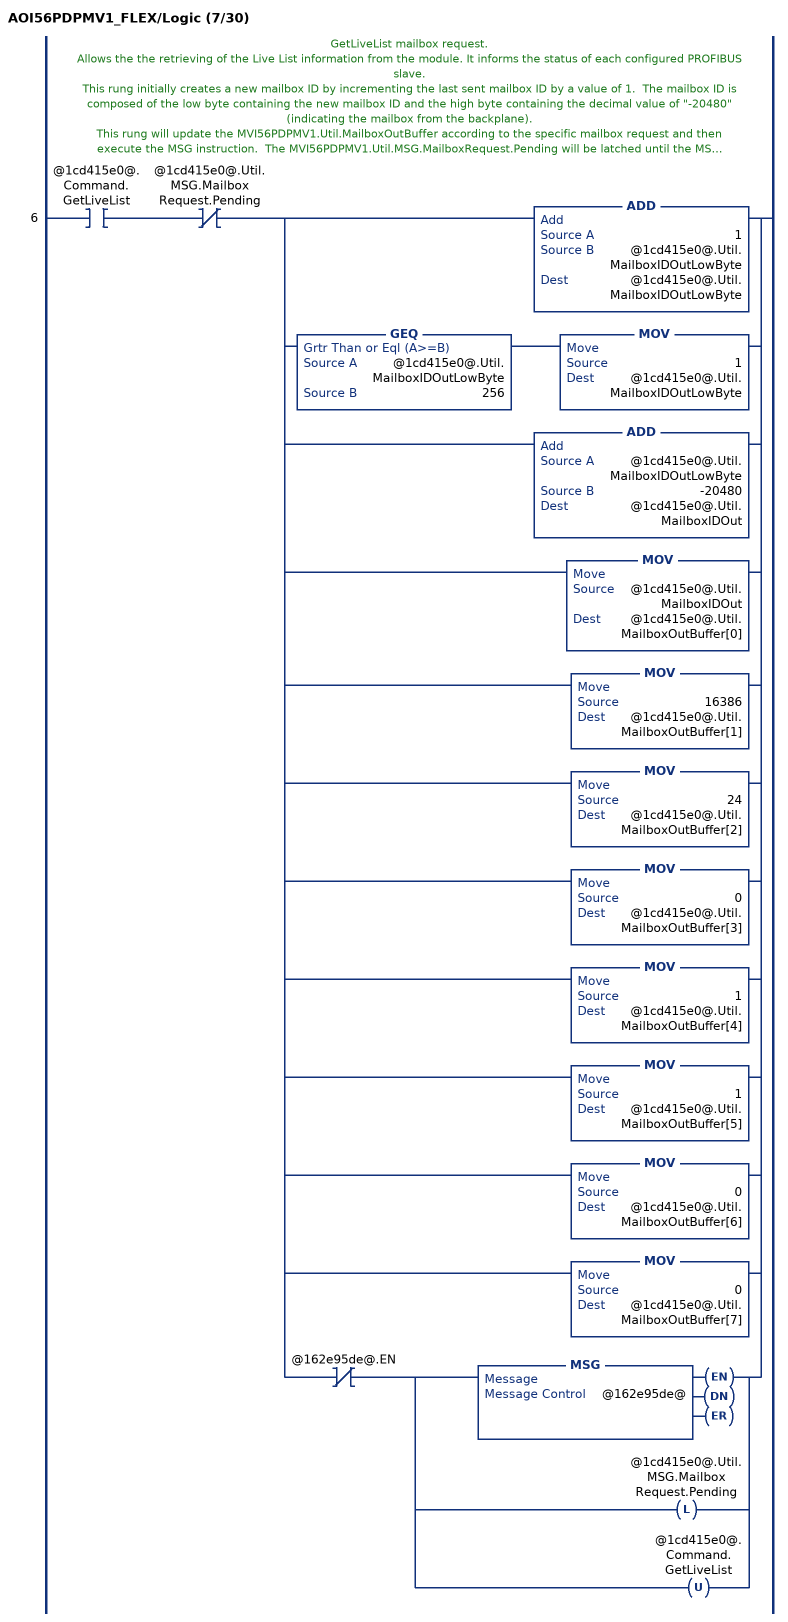
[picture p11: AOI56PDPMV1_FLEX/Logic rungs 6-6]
   // GetLiveList mailbox request.
   // Allows the the retrieving of the Live List information from the module. It informs the status of each configured PROFIBUS slave.
   // This rung initially creates a new mailbox ID by incrementing the last sent mailbox ID by a value of 1.  The mailbox ID is composed of the low byte containing the new mailbox ID and the high byte containing the decimal value of "-20480" (indicating the mailbox from the backplane).
   // This rung will update the MVI56PDPMV1.Util.MailboxOutBuffer according to the specific mailbox request and then execute the MSG instruction.  The MVI56PDPMV1.Util.MSG.MailboxRequest.Pending will be latched until the MSG operation is concluded to prevent other mailbox requests to be performed during that time. If the MSG operation is successfull then the MVI56PDPMV1.Util.MSG.MailboxRequest.DNCounter tag is incremented and the DN bit is cleared. If the MSG is not sucessfull then the MVI56PDPMV1.Util.MSG.MailboxRequest.ERCounter is incremented and the ER bit is cleared. A minimum of 100ms time should be kept between two consecutive requests for better performance, otherwise a MSG error might be returned.
   6: XIC(@1cd415e0@.Command.GetLiveList)XIO(@1cd415e0@.Util.MSG.MailboxRequest.Pending)[[ADD(1,@1cd415e0@.Util.MailboxIDOutLowByte,@1cd415e0@.Util.MailboxIDOutLowByte) ,GEQ(@1cd415e0@.Util.MailboxIDOutLowByte,256) MOV(1,@1cd415e0@.Util.MailboxIDOutLowByte) ,ADD(@1cd415e0@.Util.MailboxIDOutLowByte,-20480,@1cd415e0@.Util.MailboxIDOut) ] ,MOV(@1cd415e0@.Util.MailboxIDOut,@1cd415e0@.Util.MailboxOutBuffer[0]) ,MOV(16386,@1cd415e0@.Util.MailboxOutBuffer[1]) ,MOV(24,@1cd415e0@.Util.MailboxOutBuffer[2]) ,MOV(0,@1cd415e0@.Util.MailboxOutBuffer[3]) ,MOV(1,@1cd415e0@.Util.MailboxOutBuffer[4]) ,MOV(1,@1cd415e0@.Util.MailboxOutBuffer[5]) ,MOV(0,@1cd415e0@.Util.MailboxOutBuffer[6]) ,MOV(0,@1cd415e0@.Util.MailboxOutBuffer[7]) ,XIO(@162e95de@.EN) [MSG(@162e95de@) ,OTL(@1cd415e0@.Util.MSG.MailboxRequest.Pending) ,OTU(@1cd415e0@.Command.GetLiveList) ] ];
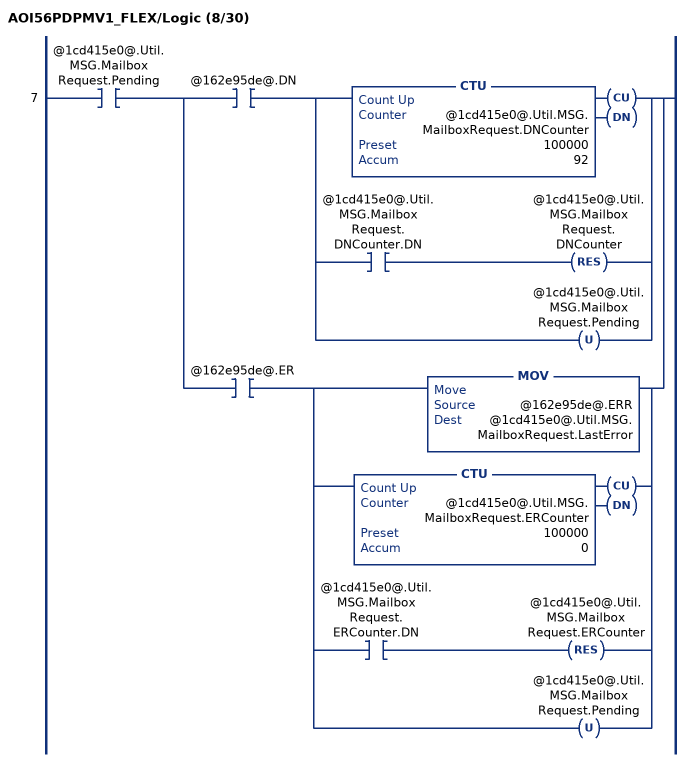
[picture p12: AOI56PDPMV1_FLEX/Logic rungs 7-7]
   7: XIC(@1cd415e0@.Util.MSG.MailboxRequest.Pending)[XIC(@162e95de@.DN) [CTU(@1cd415e0@.Util.MSG.MailboxRequest.DNCounter,100000,92) ,XIC(@1cd415e0@.Util.MSG.MailboxRequest.DNCounter.DN) RES(@1cd415e0@.Util.MSG.MailboxRequest.DNCounter) ,OTU(@1cd415e0@.Util.MSG.MailboxRequest.Pending) ] ,XIC(@162e95de@.ER) [MOV(@162e95de@.ERR,@1cd415e0@.Util.MSG.MailboxRequest.LastError) ,CTU(@1cd415e0@.Util.MSG.MailboxRequest.ERCounter,100000,0) ,XIC(@1cd415e0@.Util.MSG.MailboxRequest.ERCounter.DN) RES(@1cd415e0@.Util.MSG.MailboxRequest.ERCounter) ,OTU(@1cd415e0@.Util.MSG.MailboxRequest.Pending) ] ];
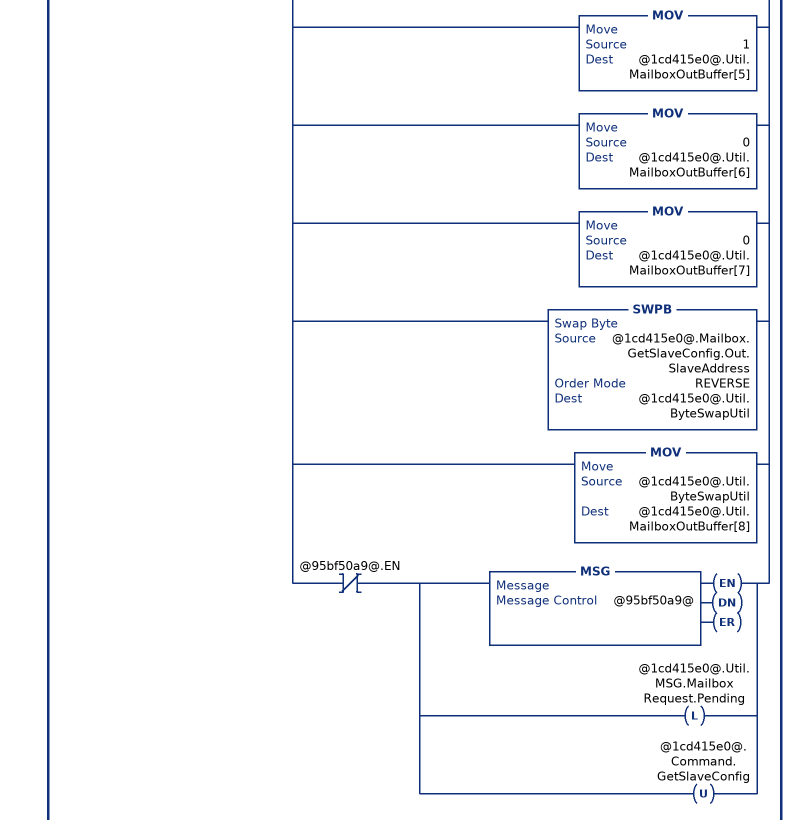
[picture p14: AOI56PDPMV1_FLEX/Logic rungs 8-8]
   // GetSlaveConfig mailbox request.
   // Allows the reading of the configuration data from a specific PROFIBUS slave.
   // This rung initially creates a new mailbox ID by incrementing the last sent mailbox ID by a value of 1.  The mailbox ID is composed of the low byte containing the new mailbox ID and the high byte containing the decimal value of "-20480" (indicating the mailbox from the backplane).
   // This rung will update the MVI56PDPMV1.Util.MailboxOutBuffer according to the specific mailbox request and then execute the MSG instruction.  The MVI56PDPMV1.Util.MSG.MailboxRequest.Pending will be latched until the MSG operation is concluded to prevent other mailbox requests to be performed during that time. If the MSG operation is successfull then the MVI56PDPMV1.Util.MSG.MailboxRequest.DNCounter tag is incremented and the DN bit is cleared. If the MSG is not sucessfull then the MVI56PDPMV1.Util.MSG.MailboxRequest.ERCounter is incremented and the ER bit is cleared. A minimum of 100ms time should be kept between two consecutive requests for better performance, otherwise a MSG error might be returned.
   8: XIC(@1cd415e0@.Command.GetSlaveConfig)XIO(@1cd415e0@.Util.MSG.MailboxRequest.Pending)[[ADD(1,@1cd415e0@.Util.MailboxIDOutLowByte,@1cd415e0@.Util.MailboxIDOutLowByte) ,GEQ(@1cd415e0@.Util.MailboxIDOutLowByte,256) MOV(1,@1cd415e0@.Util.MailboxIDOutLowByte) ,ADD(@1cd415e0@.Util.MailboxIDOutLowByte,-20480,@1cd415e0@.Util.MailboxIDOut) ] ,MOV(@1cd415e0@.Util.MailboxIDOut,@1cd415e0@.Util.MailboxOutBuffer[0]) ,MOV(16386,@1cd415e0@.Util.MailboxOutBuffer[1]) ,MOV(5,@1cd415e0@.Util.MailboxOutBuffer[2]) ,MOV(0,@1cd415e0@.Util.MailboxOutBuffer[3]) ,MOV(1,@1cd415e0@.Util.MailboxOutBuffer[4]) ,MOV(1,@1cd415e0@.Util.MailboxOutBuffer[5]) ,MOV(0,@1cd415e0@.Util.MailboxOutBuffer[6]) ,MOV(0,@1cd415e0@.Util.MailboxOutBuffer[7]) ,SWPB(@1cd415e0@.Mailbox.GetSlaveConfig.Out.SlaveAddress,REVERSE,@1cd415e0@.Util.ByteSwapUtil) ,MOV(@1cd415e0@.Util.ByteSwapUtil,@1cd415e0@.Util.MailboxOutBuffer[8]) ,XIO(@95bf50a9@.EN) [MSG(@95bf50a9@) ,OTL(@1cd415e0@.Util.MSG.MailboxRequest.Pending) ,OTU(@1cd415e0@.Command.GetSlaveConfig) ] ];
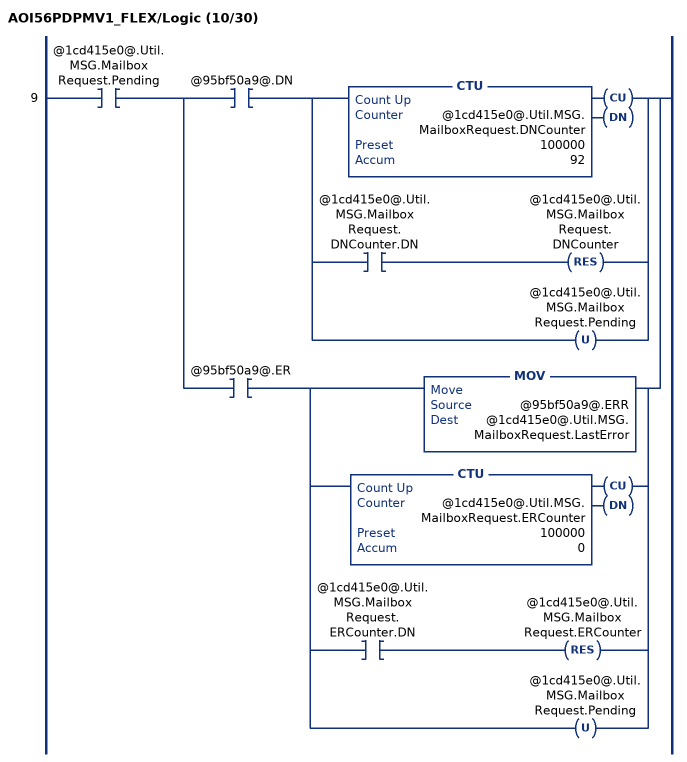
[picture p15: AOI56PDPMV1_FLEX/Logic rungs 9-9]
   9: XIC(@1cd415e0@.Util.MSG.MailboxRequest.Pending)[XIC(@95bf50a9@.DN) [CTU(@1cd415e0@.Util.MSG.MailboxRequest.DNCounter,100000,92) ,XIC(@1cd415e0@.Util.MSG.MailboxRequest.DNCounter.DN) RES(@1cd415e0@.Util.MSG.MailboxRequest.DNCounter) ,OTU(@1cd415e0@.Util.MSG.MailboxRequest.Pending) ] ,XIC(@95bf50a9@.ER) [MOV(@95bf50a9@.ERR,@1cd415e0@.Util.MSG.MailboxRequest.LastError) ,CTU(@1cd415e0@.Util.MSG.MailboxRequest.ERCounter,100000,0) ,XIC(@1cd415e0@.Util.MSG.MailboxRequest.ERCounter.DN) RES(@1cd415e0@.Util.MSG.MailboxRequest.ERCounter) ,OTU(@1cd415e0@.Util.MSG.MailboxRequest.Pending) ] ];
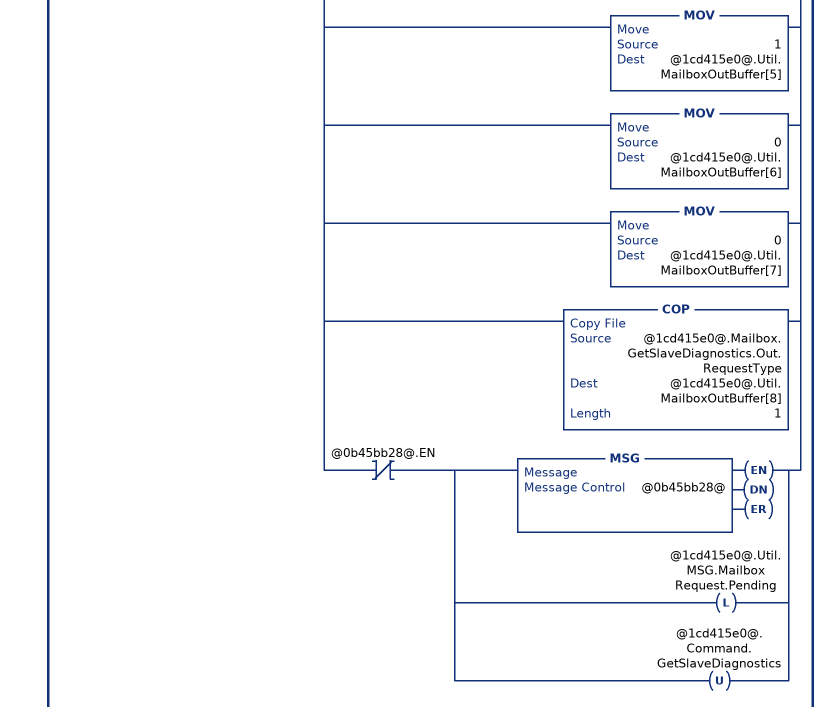
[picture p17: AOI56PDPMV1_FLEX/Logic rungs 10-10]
   // GetSlaveDiagnostics mailbox request.
   // Allows the reading of extended diagnostic information from a specific PROFIBUS slave.
   // This rung initially creates a new mailbox ID by incrementing the last sent mailbox ID by a value of 1.  The mailbox ID is composed of the low byte containing the new mailbox ID and the high byte containing the decimal value of "-20480" (indicating the mailbox from the backplane).
   // This rung will update the MVI56PDPMV1.Util.MailboxOutBuffer according to the specific mailbox request and then execute the MSG instruction.  The MVI56PDPMV1.Util.MSG.MailboxRequest.Pending will be latched until the MSG operation is concluded to prevent other mailbox requests to be performed during that time. If the MSG operation is successfull then the MVI56PDPMV1.Util.MSG.MailboxRequest.DNCounter tag is incremented and the DN bit is cleared. If the MSG is not sucessfull then the MVI56PDPMV1.Util.MSG.MailboxRequest.ERCounter is incremented and the ER bit is cleared. A minimum of 100ms time should be kept between two consecutive requests for better performance, otherwise a MSG error might be returned.
   10: XIC(@1cd415e0@.Command.GetSlaveDiagnostics)XIO(@1cd415e0@.Util.MSG.MailboxRequest.Pending)[[ADD(1,@1cd415e0@.Util.MailboxIDOutLowByte,@1cd415e0@.Util.MailboxIDOutLowByte) ,GEQ(@1cd415e0@.Util.MailboxIDOutLowByte,256) MOV(1,@1cd415e0@.Util.MailboxIDOutLowByte) ,ADD(@1cd415e0@.Util.MailboxIDOutLowByte,-20480,@1cd415e0@.Util.MailboxIDOut) ] ,MOV(@1cd415e0@.Util.MailboxIDOut,@1cd415e0@.Util.MailboxOutBuffer[0]) ,MOV(16386,@1cd415e0@.Util.MailboxOutBuffer[1]) ,MOV(4,@1cd415e0@.Util.MailboxOutBuffer[2]) ,MOV(0,@1cd415e0@.Util.MailboxOutBuffer[3]) ,MOV(1,@1cd415e0@.Util.MailboxOutBuffer[4]) ,MOV(1,@1cd415e0@.Util.MailboxOutBuffer[5]) ,MOV(0,@1cd415e0@.Util.MailboxOutBuffer[6]) ,MOV(0,@1cd415e0@.Util.MailboxOutBuffer[7]) ,COP(@1cd415e0@.Mailbox.GetSlaveDiagnostics.Out.RequestType,@1cd415e0@.Util.MailboxOutBuffer[8],1) ,XIO(@0b45bb28@.EN) [MSG(@0b45bb28@) ,OTL(@1cd415e0@.Util.MSG.MailboxRequest.Pending) ,OTU(@1cd415e0@.Command.GetSlaveDiagnostics) ] ];
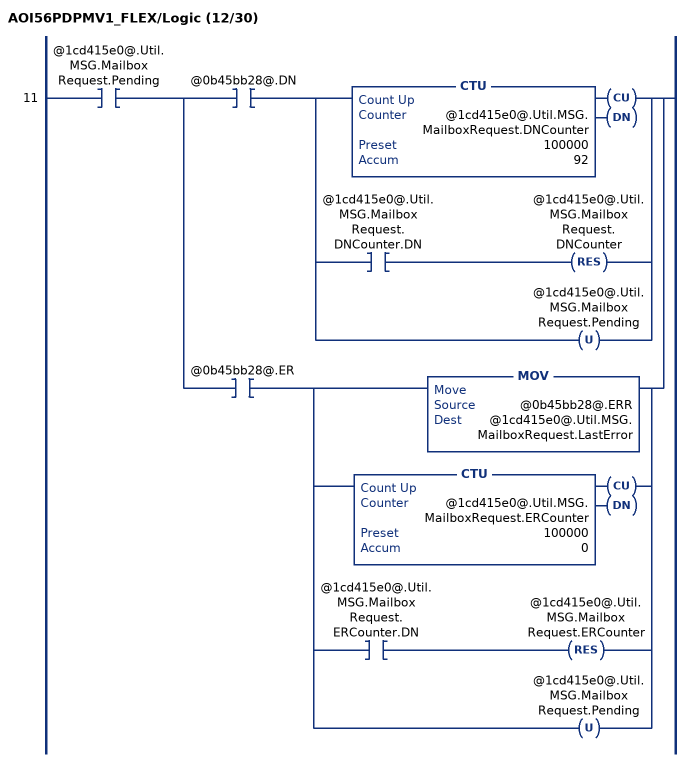
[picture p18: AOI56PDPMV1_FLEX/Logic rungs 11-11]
   11: XIC(@1cd415e0@.Util.MSG.MailboxRequest.Pending)[XIC(@0b45bb28@.DN) [CTU(@1cd415e0@.Util.MSG.MailboxRequest.DNCounter,100000,92) ,XIC(@1cd415e0@.Util.MSG.MailboxRequest.DNCounter.DN) RES(@1cd415e0@.Util.MSG.MailboxRequest.DNCounter) ,OTU(@1cd415e0@.Util.MSG.MailboxRequest.Pending) ] ,XIC(@0b45bb28@.ER) [MOV(@0b45bb28@.ERR,@1cd415e0@.Util.MSG.MailboxRequest.LastError) ,CTU(@1cd415e0@.Util.MSG.MailboxRequest.ERCounter,100000,0) ,XIC(@1cd415e0@.Util.MSG.MailboxRequest.ERCounter.DN) RES(@1cd415e0@.Util.MSG.MailboxRequest.ERCounter) ,OTU(@1cd415e0@.Util.MSG.MailboxRequest.Pending) ] ];
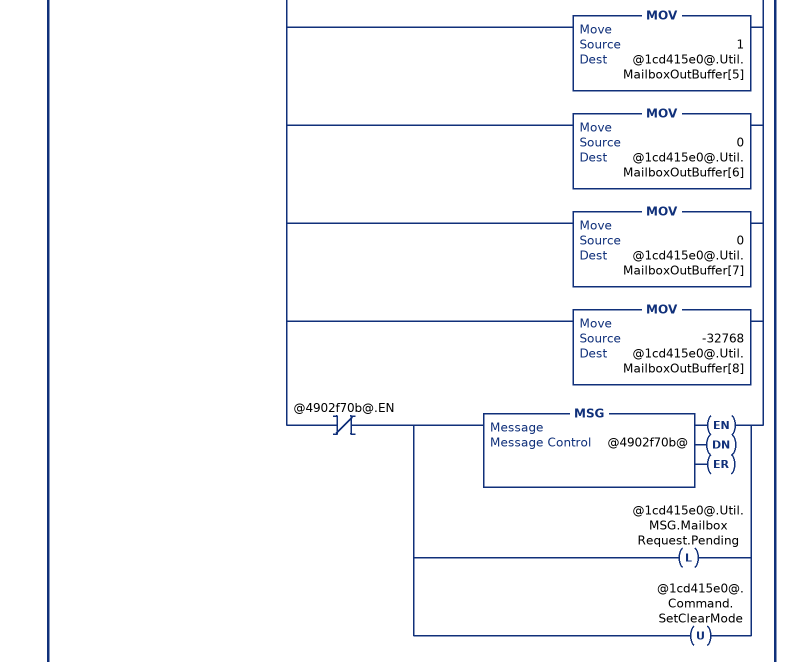
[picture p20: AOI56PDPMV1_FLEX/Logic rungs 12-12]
   // SetClearMode mailbox request.
   // Allows the processor to change the module into clear mode (no PROFIBUS output update, only PROFIBUS input will be read into the module).
   // This rung initially creates a new mailbox ID by incrementing the last sent mailbox ID by a value of 1.  The mailbox ID is composed of the low byte containing the new mailbox ID and the high byte containing the decimal value of "-20480" (indicating the mailbox from the backplane).
   // This rung will update the MVI56PDPMV1.Util.MailboxOutBuffer according to the specific mailbox request and then execute the MSG instruction.  The MVI56PDPMV1.Util.MSG.MailboxRequest.Pending will be latched until the MSG operation is concluded to prevent other mailbox requests to be performed during that time. If the MSG operation is successfull then the MVI56PDPMV1.Util.MSG.MailboxRequest.DNCounter tag is incremented and the DN bit is cleared. If the MSG is not sucessfull then the MVI56PDPMV1.Util.MSG.MailboxRequest.ERCounter is incremented and the ER bit is cleared. A minimum of 100ms time should be kept between two consecutive requests for better performance, otherwise a MSG error might be returned.
   12: XIC(@1cd415e0@.Command.SetClearMode)XIO(@1cd415e0@.Util.MSG.MailboxRequest.Pending)[[ADD(1,@1cd415e0@.Util.MailboxIDOutLowByte,@1cd415e0@.Util.MailboxIDOutLowByte) ,GEQ(@1cd415e0@.Util.MailboxIDOutLowByte,256) MOV(1,@1cd415e0@.Util.MailboxIDOutLowByte) ,ADD(@1cd415e0@.Util.MailboxIDOutLowByte,-20480,@1cd415e0@.Util.MailboxIDOut) ] ,MOV(@1cd415e0@.Util.MailboxIDOut,@1cd415e0@.Util.MailboxOutBuffer[0]) ,MOV(16386,@1cd415e0@.Util.MailboxOutBuffer[1]) ,MOV(2,@1cd415e0@.Util.MailboxOutBuffer[2]) ,MOV(0,@1cd415e0@.Util.MailboxOutBuffer[3]) ,MOV(1,@1cd415e0@.Util.MailboxOutBuffer[4]) ,MOV(1,@1cd415e0@.Util.MailboxOutBuffer[5]) ,MOV(0,@1cd415e0@.Util.MailboxOutBuffer[6]) ,MOV(0,@1cd415e0@.Util.MailboxOutBuffer[7]) ,MOV(-32768,@1cd415e0@.Util.MailboxOutBuffer[8]) ,XIO(@4902f70b@.EN) [MSG(@4902f70b@) ,OTL(@1cd415e0@.Util.MSG.MailboxRequest.Pending) ,OTU(@1cd415e0@.Command.SetClearMode) ] ];
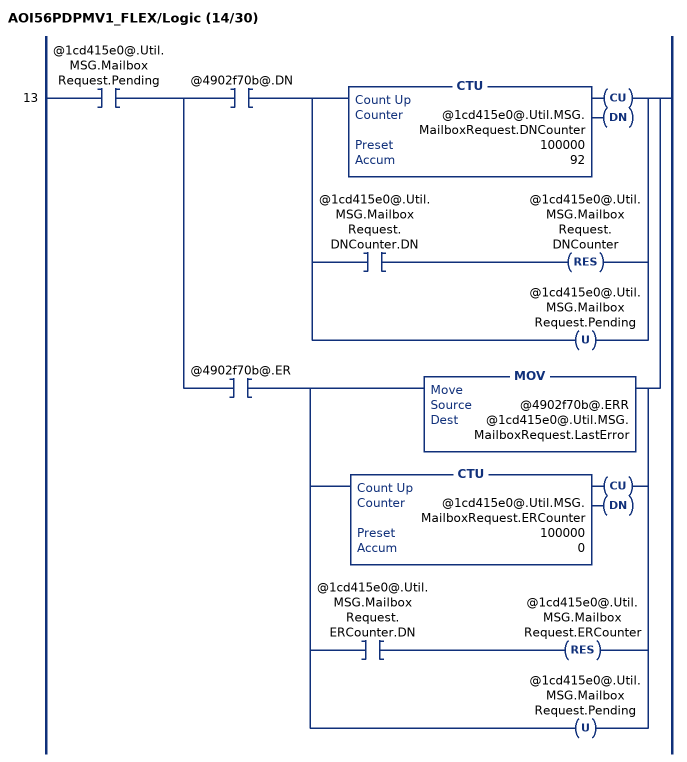
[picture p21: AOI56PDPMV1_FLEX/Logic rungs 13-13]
   13: XIC(@1cd415e0@.Util.MSG.MailboxRequest.Pending)[XIC(@4902f70b@.DN) [CTU(@1cd415e0@.Util.MSG.MailboxRequest.DNCounter,100000,92) ,XIC(@1cd415e0@.Util.MSG.MailboxRequest.DNCounter.DN) RES(@1cd415e0@.Util.MSG.MailboxRequest.DNCounter) ,OTU(@1cd415e0@.Util.MSG.MailboxRequest.Pending) ] ,XIC(@4902f70b@.ER) [MOV(@4902f70b@.ERR,@1cd415e0@.Util.MSG.MailboxRequest.LastError) ,CTU(@1cd415e0@.Util.MSG.MailboxRequest.ERCounter,100000,0) ,XIC(@1cd415e0@.Util.MSG.MailboxRequest.ERCounter.DN) RES(@1cd415e0@.Util.MSG.MailboxRequest.ERCounter) ,OTU(@1cd415e0@.Util.MSG.MailboxRequest.Pending) ] ];
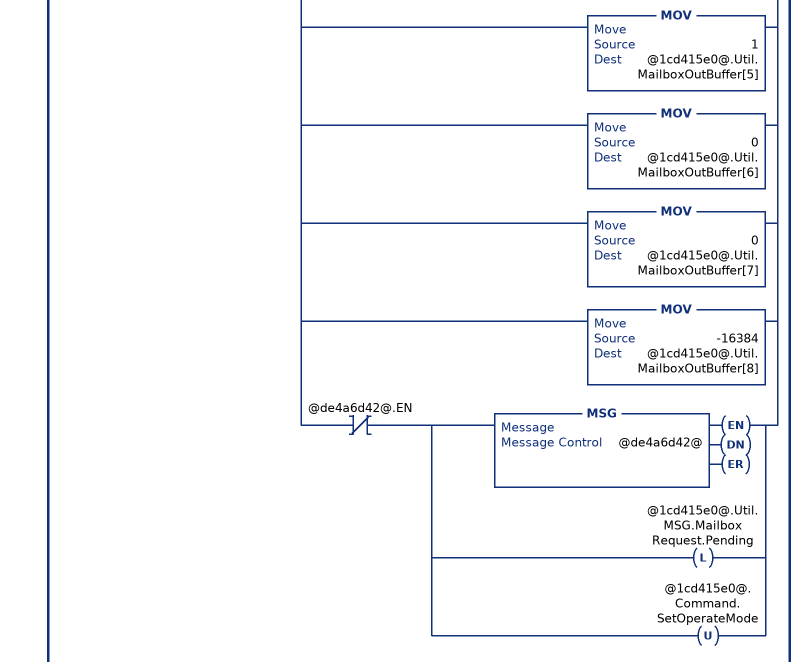
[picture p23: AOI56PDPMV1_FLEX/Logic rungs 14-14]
   // SetOperateMode mailbox request.
   // The module will only update I/O in operate mode. The module is initialized in operate mode, but it can be changed to Clear or Operate modes through mailbox requests.
   // This rung initially creates a new mailbox ID by incrementing the last sent mailbox ID by a value of 1.  The mailbox ID is composed of the low byte containing the new mailbox ID and the high byte containing the decimal value of "-20480" (indicating the mailbox from the backplane).
   // This rung will update the MVI56PDPMV1.Util.MailboxOutBuffer according to the specific mailbox request and then execute the MSG instruction.  The MVI56PDPMV1.Util.MSG.MailboxRequest.Pending will be latched until the MSG operation is concluded to prevent other mailbox requests to be performed during that time. If the MSG operation is successfull then the MVI56PDPMV1.Util.MSG.MailboxRequest.DNCounter tag is incremented and the DN bit is cleared. If the MSG is not sucessfull then the MVI56PDPMV1.Util.MSG.MailboxRequest.ERCounter is incremented and the ER bit is cleared. A minimum of 100ms time should be kept between two consecutive requests for better performance, otherwise a MSG error might be returned.
   14: XIC(@1cd415e0@.Command.SetOperateMode)XIO(@1cd415e0@.Util.MSG.MailboxRequest.Pending)[[ADD(1,@1cd415e0@.Util.MailboxIDOutLowByte,@1cd415e0@.Util.MailboxIDOutLowByte) ,GEQ(@1cd415e0@.Util.MailboxIDOutLowByte,256) MOV(1,@1cd415e0@.Util.MailboxIDOutLowByte) ,ADD(@1cd415e0@.Util.MailboxIDOutLowByte,-20480,@1cd415e0@.Util.MailboxIDOut) ] ,MOV(@1cd415e0@.Util.MailboxIDOut,@1cd415e0@.Util.MailboxOutBuffer[0]) ,MOV(16386,@1cd415e0@.Util.MailboxOutBuffer[1]) ,MOV(2,@1cd415e0@.Util.MailboxOutBuffer[2]) ,MOV(0,@1cd415e0@.Util.MailboxOutBuffer[3]) ,MOV(1,@1cd415e0@.Util.MailboxOutBuffer[4]) ,MOV(1,@1cd415e0@.Util.MailboxOutBuffer[5]) ,MOV(0,@1cd415e0@.Util.MailboxOutBuffer[6]) ,MOV(0,@1cd415e0@.Util.MailboxOutBuffer[7]) ,MOV(-16384,@1cd415e0@.Util.MailboxOutBuffer[8]) ,XIO(@de4a6d42@.EN) [MSG(@de4a6d42@) ,OTL(@1cd415e0@.Util.MSG.MailboxRequest.Pending) ,OTU(@1cd415e0@.Command.SetOperateMode) ] ];
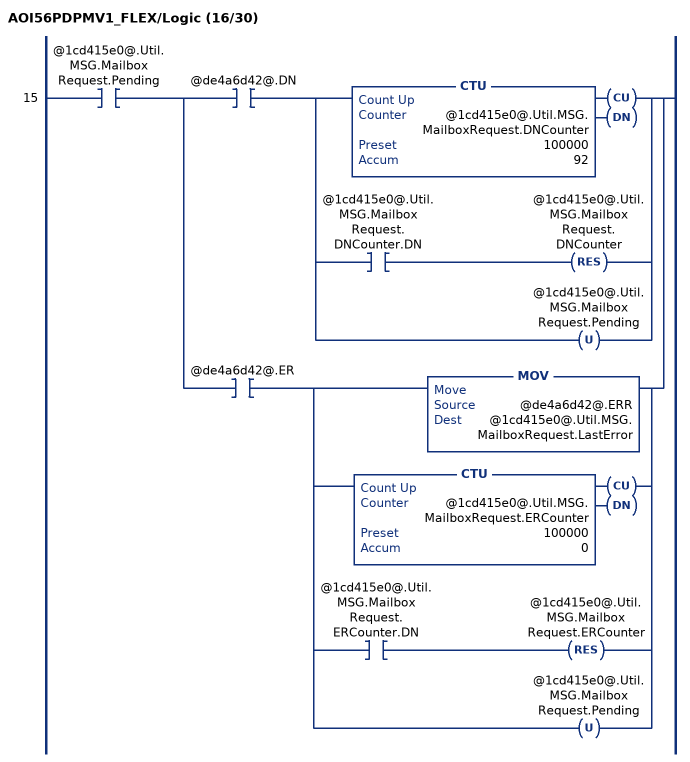
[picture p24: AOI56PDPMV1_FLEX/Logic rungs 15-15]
   15: XIC(@1cd415e0@.Util.MSG.MailboxRequest.Pending)[XIC(@de4a6d42@.DN) [CTU(@1cd415e0@.Util.MSG.MailboxRequest.DNCounter,100000,92) ,XIC(@1cd415e0@.Util.MSG.MailboxRequest.DNCounter.DN) RES(@1cd415e0@.Util.MSG.MailboxRequest.DNCounter) ,OTU(@1cd415e0@.Util.MSG.MailboxRequest.Pending) ] ,XIC(@de4a6d42@.ER) [MOV(@de4a6d42@.ERR,@1cd415e0@.Util.MSG.MailboxRequest.LastError) ,CTU(@1cd415e0@.Util.MSG.MailboxRequest.ERCounter,100000,0) ,XIC(@1cd415e0@.Util.MSG.MailboxRequest.ERCounter.DN) RES(@1cd415e0@.Util.MSG.MailboxRequest.ERCounter) ,OTU(@1cd415e0@.Util.MSG.MailboxRequest.Pending) ] ];
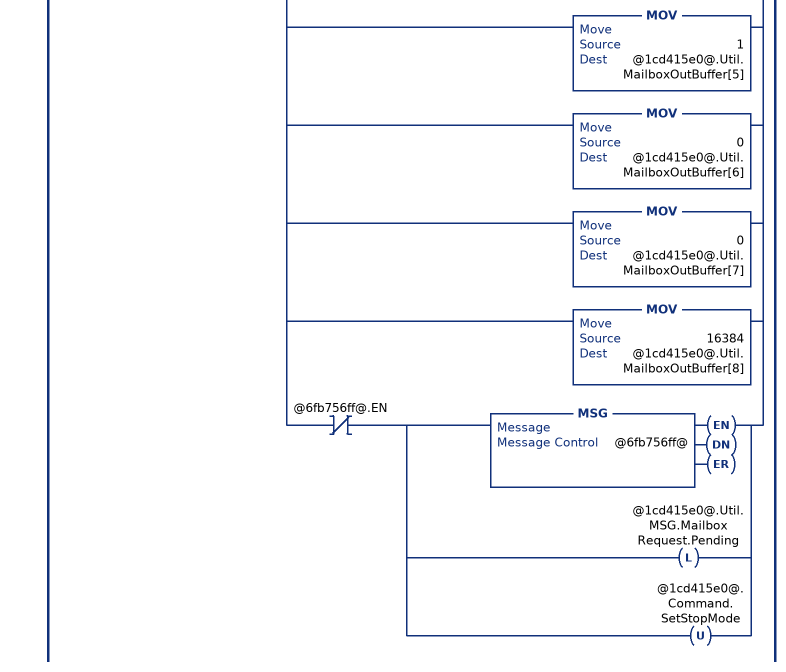
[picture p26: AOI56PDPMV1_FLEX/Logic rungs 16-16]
   // SetStopMode mailbox request.
   // The module will not communicate to any PROFIBUS slaves while in stop mode.
   // This rung initially creates a new mailbox ID by incrementing the last sent mailbox ID by a value of 1.  The mailbox ID is composed of the low byte containing the new mailbox ID and the high byte containing the decimal value of "-20480" (indicating the mailbox from the backplane).
   // This rung will update the MVI56PDPMV1.Util.MailboxOutBuffer according to the specific mailbox request and then execute the MSG instruction.  The MVI56PDPMV1.Util.MSG.MailboxRequest.Pending will be latched until the MSG operation is concluded to prevent other mailbox requests to be performed during that time. If the MSG operation is successfull then the MVI56PDPMV1.Util.MSG.MailboxRequest.DNCounter tag is incremented and the DN bit is cleared. If the MSG is not sucessfull then the MVI56PDPMV1.Util.MSG.MailboxRequest.ERCounter is incremented and the ER bit is cleared. A minimum of 100ms time should be kept between two consecutive requests for better performance, otherwise a MSG error might be returned.
   16: XIC(@1cd415e0@.Command.SetStopMode)XIO(@1cd415e0@.Util.MSG.MailboxRequest.Pending)[[ADD(1,@1cd415e0@.Util.MailboxIDOutLowByte,@1cd415e0@.Util.MailboxIDOutLowByte) ,GEQ(@1cd415e0@.Util.MailboxIDOutLowByte,256) MOV(1,@1cd415e0@.Util.MailboxIDOutLowByte) ,ADD(@1cd415e0@.Util.MailboxIDOutLowByte,-20480,@1cd415e0@.Util.MailboxIDOut) ] ,MOV(@1cd415e0@.Util.MailboxIDOut,@1cd415e0@.Util.MailboxOutBuffer[0]) ,MOV(16386,@1cd415e0@.Util.MailboxOutBuffer[1]) ,MOV(2,@1cd415e0@.Util.MailboxOutBuffer[2]) ,MOV(0,@1cd415e0@.Util.MailboxOutBuffer[3]) ,MOV(1,@1cd415e0@.Util.MailboxOutBuffer[4]) ,MOV(1,@1cd415e0@.Util.MailboxOutBuffer[5]) ,MOV(0,@1cd415e0@.Util.MailboxOutBuffer[6]) ,MOV(0,@1cd415e0@.Util.MailboxOutBuffer[7]) ,MOV(16384,@1cd415e0@.Util.MailboxOutBuffer[8]) ,XIO(@6fb756ff@.EN) [MSG(@6fb756ff@) ,OTL(@1cd415e0@.Util.MSG.MailboxRequest.Pending) ,OTU(@1cd415e0@.Command.SetStopMode) ] ];
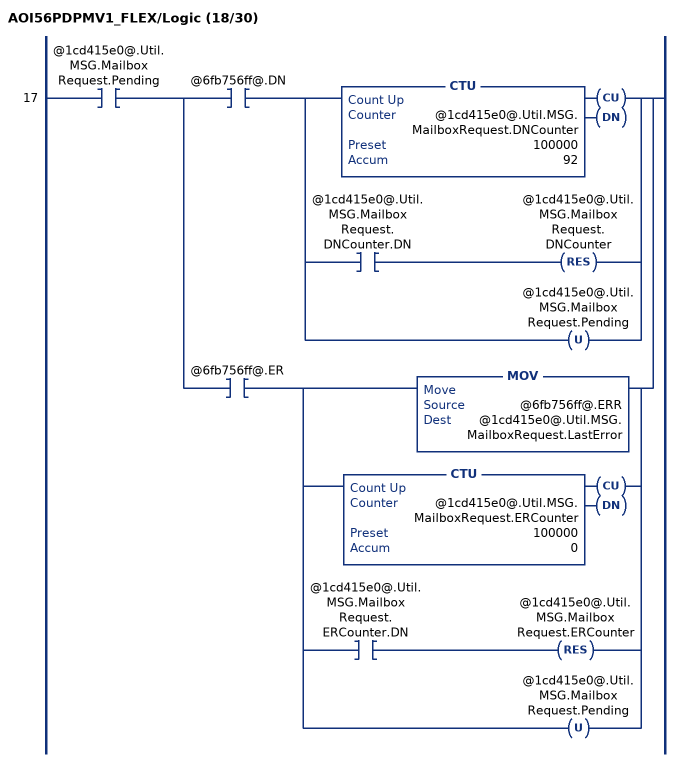
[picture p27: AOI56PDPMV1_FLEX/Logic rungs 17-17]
   17: XIC(@1cd415e0@.Util.MSG.MailboxRequest.Pending)[XIC(@6fb756ff@.DN) [CTU(@1cd415e0@.Util.MSG.MailboxRequest.DNCounter,100000,92) ,XIC(@1cd415e0@.Util.MSG.MailboxRequest.DNCounter.DN) RES(@1cd415e0@.Util.MSG.MailboxRequest.DNCounter) ,OTU(@1cd415e0@.Util.MSG.MailboxRequest.Pending) ] ,XIC(@6fb756ff@.ER) [MOV(@6fb756ff@.ERR,@1cd415e0@.Util.MSG.MailboxRequest.LastError) ,CTU(@1cd415e0@.Util.MSG.MailboxRequest.ERCounter,100000,0) ,XIC(@1cd415e0@.Util.MSG.MailboxRequest.ERCounter.DN) RES(@1cd415e0@.Util.MSG.MailboxRequest.ERCounter) ,OTU(@1cd415e0@.Util.MSG.MailboxRequest.Pending) ] ];
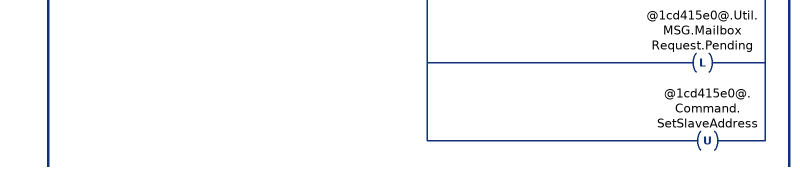
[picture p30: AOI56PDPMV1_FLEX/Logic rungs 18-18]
   // SetSlaveAddress mailbox request.
   // Sends a mailbox request to dynamically change the PROFIBUS address of a specific slave. Only certain slaves will support this funcionality.
   // This rung initially creates a new mailbox ID by incrementing the last sent mailbox ID by a value of 1.  The mailbox ID is composed of the low byte containing the new mailbox ID and the high byte containing the decimal value of "-20480" (indicating the mailbox from the backplane).
   // This rung will update the MVI56PDPMV1.Util.MailboxOutBuffer according to the specific mailbox request and then execute the MSG instruction.  The MVI56PDPMV1.Util.MSG.MailboxRequest.Pending will be latched until the MSG operation is concluded to prevent other mailbox requests to be performed during that time. If the MSG operation is successfull then the MVI56PDPMV1.Util.MSG.MailboxRequest.DNCounter tag is incremented and the DN bit is cleared. If the MSG is not sucessfull then the MVI56PDPMV1.Util.MSG.MailboxRequest.ERCounter is incremented and the ER bit is cleared. A minimum of 100ms time should be kept between two consecutive requests for better performance, otherwise a MSG error might be returned.
   18: XIC(@1cd415e0@.Command.SetSlaveAddress)XIO(@1cd415e0@.Util.MSG.MailboxRequest.Pending)[[ADD(1,@1cd415e0@.Util.MailboxIDOutLowByte,@1cd415e0@.Util.MailboxIDOutLowByte) ,GEQ(@1cd415e0@.Util.MailboxIDOutLowByte,256) MOV(1,@1cd415e0@.Util.MailboxIDOutLowByte) ,ADD(@1cd415e0@.Util.MailboxIDOutLowByte,-20480,@1cd415e0@.Util.MailboxIDOut) ] ,MOV(@1cd415e0@.Util.MailboxIDOut,@1cd415e0@.Util.MailboxOutBuffer[0]) ,MOV(16386,@1cd415e0@.Util.MailboxOutBuffer[1]) ,MOV(6,@1cd415e0@.Util.MailboxOutBuffer[2]) ,MOV(@1cd415e0@.Mailbox.SetSlaveAddress.Out.ByteCount,@1cd415e0@.Util.MailboxOutBuffer[3]) ,MOV(1,@1cd415e0@.Util.MailboxOutBuffer[4]) ,MOV(1,@1cd415e0@.Util.MailboxOutBuffer[5]) ,MOV(0,@1cd415e0@.Util.MailboxOutBuffer[6]) ,MOV(0,@1cd415e0@.Util.MailboxOutBuffer[7]) ,COP(@1cd415e0@.Mailbox.SetSlaveAddress.Out.NewSlaveAddress,@1cd415e0@.Util.MailboxOutBuffer[8],1) ,MOV(@1cd415e0@.Mailbox.SetSlaveAddress.Out.SlaveIdentNumber,@1cd415e0@.Util.MailboxOutBuffer[9]) ,SWPB(@1cd415e0@.Mailbox.SetSlaveAddress.Out.No_add_Chg,REVERSE,@1cd415e0@.Util.ByteSwapUtil) ,MOV(@1cd415e0@.Util.ByteSwapUtil,@1cd415e0@.Util.MailboxOutBuffer[10]) ,COP(@1cd415e0@.Mailbox.SetSlaveAddress.In.MessageDataByte[0],@1cd415e0@.Util.MailboxOutBuffer[16],100) ,XIO(@d93638fd@.EN) [MSG(@d93638fd@) ,OTL(@1cd415e0@.Util.MSG.MailboxRequest.Pending) ,OTU(@1cd415e0@.Command.SetSlaveAddress) ] ];
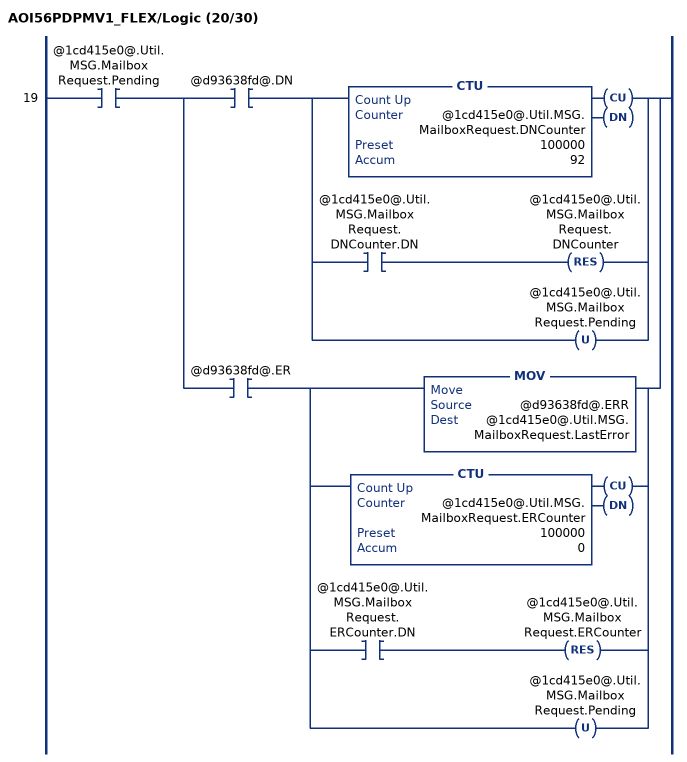
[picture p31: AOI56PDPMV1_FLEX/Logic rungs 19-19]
   19: XIC(@1cd415e0@.Util.MSG.MailboxRequest.Pending)[XIC(@d93638fd@.DN) [CTU(@1cd415e0@.Util.MSG.MailboxRequest.DNCounter,100000,92) ,XIC(@1cd415e0@.Util.MSG.MailboxRequest.DNCounter.DN) RES(@1cd415e0@.Util.MSG.MailboxRequest.DNCounter) ,OTU(@1cd415e0@.Util.MSG.MailboxRequest.Pending) ] ,XIC(@d93638fd@.ER) [MOV(@d93638fd@.ERR,@1cd415e0@.Util.MSG.MailboxRequest.LastError) ,CTU(@1cd415e0@.Util.MSG.MailboxRequest.ERCounter,100000,0) ,XIC(@1cd415e0@.Util.MSG.MailboxRequest.ERCounter.DN) RES(@1cd415e0@.Util.MSG.MailboxRequest.ERCounter) ,OTU(@1cd415e0@.Util.MSG.MailboxRequest.Pending) ] ];
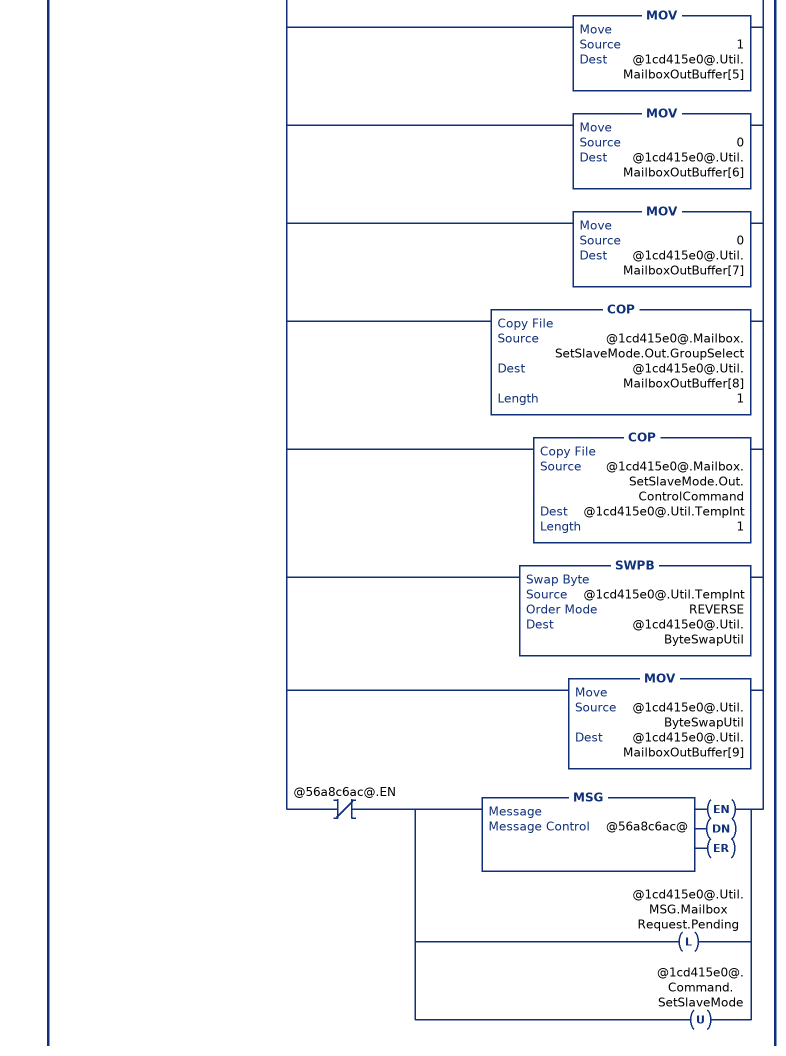
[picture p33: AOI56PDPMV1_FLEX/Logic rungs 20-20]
   // SetSlaveMode mailbox request.
   // This mailbox allows the processor to change certain slaves or group of slaves to sync or freeze mode. Check documentation for further details.
   // This rung initially creates a new mailbox ID by incrementing the last sent mailbox ID by a value of 1.  The mailbox ID is composed of the low byte containing the new mailbox ID and the high byte containing the decimal value of "-20480" (indicating the mailbox from the backplane).
   // This rung will update the MVI56PDPMV1.Util.MailboxOutBuffer according to the specific mailbox request and then execute the MSG instruction.  The MVI56PDPMV1.Util.MSG.MailboxRequest.Pending will be latched until the MSG operation is concluded to prevent other mailbox requests to be performed during that time. If the MSG operation is successfull then the MVI56PDPMV1.Util.MSG.MailboxRequest.DNCounter tag is incremented and the DN bit is cleared. If the MSG is not sucessfull then the MVI56PDPMV1.Util.MSG.MailboxRequest.ERCounter is incremented and the ER bit is cleared. A minimum of 100ms time should be kept between two consecutive requests for better performance, otherwise a MSG error might be returned.
   20: XIC(@1cd415e0@.Command.SetSlaveMode)XIO(@1cd415e0@.Util.MSG.MailboxRequest.Pending)[[ADD(1,@1cd415e0@.Util.MailboxIDOutLowByte,@1cd415e0@.Util.MailboxIDOutLowByte) ,GEQ(@1cd415e0@.Util.MailboxIDOutLowByte,256) MOV(1,@1cd415e0@.Util.MailboxIDOutLowByte) ,ADD(@1cd415e0@.Util.MailboxIDOutLowByte,-20480,@1cd415e0@.Util.MailboxIDOut) ] ,MOV(@1cd415e0@.Util.MailboxIDOut,@1cd415e0@.Util.MailboxOutBuffer[0]) ,MOV(16386,@1cd415e0@.Util.MailboxOutBuffer[1]) ,MOV(3,@1cd415e0@.Util.MailboxOutBuffer[2]) ,MOV(0,@1cd415e0@.Util.MailboxOutBuffer[3]) ,MOV(1,@1cd415e0@.Util.MailboxOutBuffer[4]) ,MOV(1,@1cd415e0@.Util.MailboxOutBuffer[5]) ,MOV(0,@1cd415e0@.Util.MailboxOutBuffer[6]) ,MOV(0,@1cd415e0@.Util.MailboxOutBuffer[7]) ,COP(@1cd415e0@.Mailbox.SetSlaveMode.Out.GroupSelect,@1cd415e0@.Util.MailboxOutBuffer[8],1) ,COP(@1cd415e0@.Mailbox.SetSlaveMode.Out.ControlCommand,@1cd415e0@.Util.TempInt,1) ,SWPB(@1cd415e0@.Util.TempInt,REVERSE,@1cd415e0@.Util.ByteSwapUtil) ,MOV(@1cd415e0@.Util.ByteSwapUtil,@1cd415e0@.Util.MailboxOutBuffer[9]) ,XIO(@56a8c6ac@.EN) [MSG(@56a8c6ac@) ,OTL(@1cd415e0@.Util.MSG.MailboxRequest.Pending) ,OTU(@1cd415e0@.Command.SetSlaveMode) ] ];
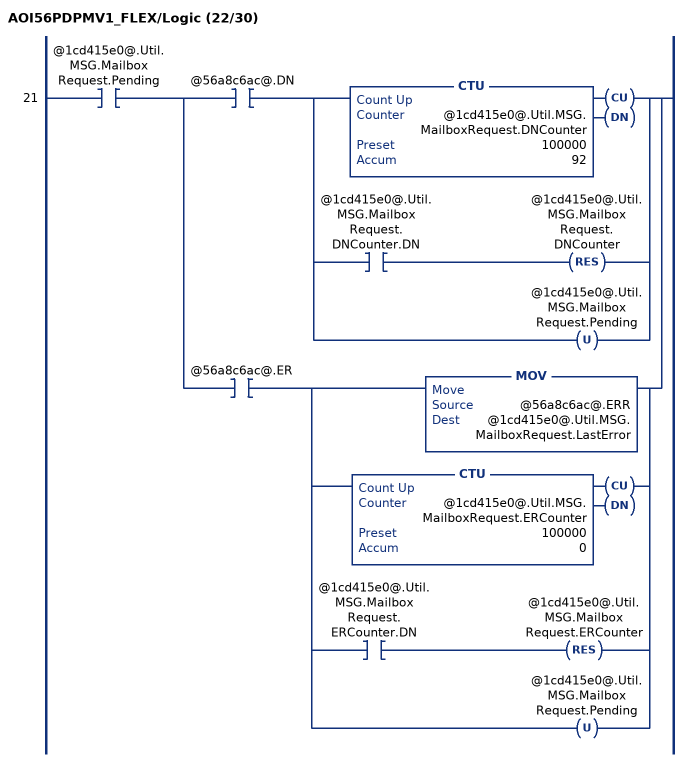
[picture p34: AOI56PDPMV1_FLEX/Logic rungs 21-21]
   21: XIC(@1cd415e0@.Util.MSG.MailboxRequest.Pending)[XIC(@56a8c6ac@.DN) [CTU(@1cd415e0@.Util.MSG.MailboxRequest.DNCounter,100000,92) ,XIC(@1cd415e0@.Util.MSG.MailboxRequest.DNCounter.DN) RES(@1cd415e0@.Util.MSG.MailboxRequest.DNCounter) ,OTU(@1cd415e0@.Util.MSG.MailboxRequest.Pending) ] ,XIC(@56a8c6ac@.ER) [MOV(@56a8c6ac@.ERR,@1cd415e0@.Util.MSG.MailboxRequest.LastError) ,CTU(@1cd415e0@.Util.MSG.MailboxRequest.ERCounter,100000,0) ,XIC(@1cd415e0@.Util.MSG.MailboxRequest.ERCounter.DN) RES(@1cd415e0@.Util.MSG.MailboxRequest.ERCounter) ,OTU(@1cd415e0@.Util.MSG.MailboxRequest.Pending) ] ];
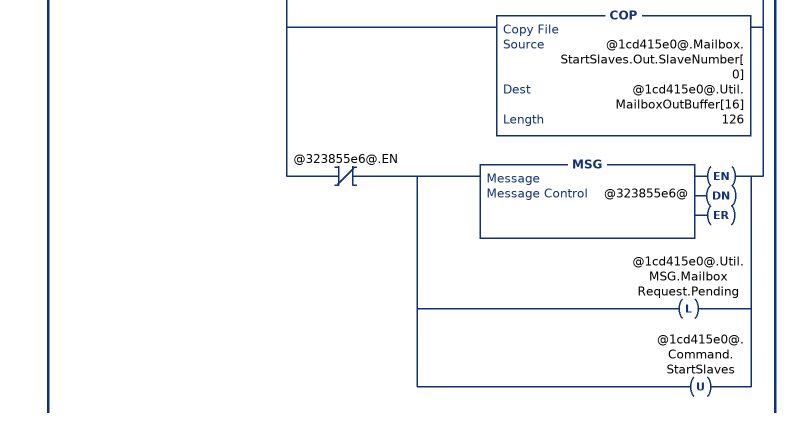
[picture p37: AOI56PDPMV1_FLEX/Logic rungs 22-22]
   // StartSlaves mailbox request.
   // This mailbox allows the restart of communication to a specific slave (after being stopped by the StopSlaves mailbox).
   // This rung initially creates a new mailbox ID by incrementing the last sent mailbox ID by a value of 1.  The mailbox ID is composed of the low byte containing the new mailbox ID and the high byte containing the decimal value of "-20480" (indicating the mailbox from the backplane).
   // This rung will update the MVI56PDPMV1.Util.MailboxOutBuffer according to the specific mailbox request and then execute the MSG instruction.  The MVI56PDPMV1.Util.MSG.MailboxRequest.Pending will be latched until the MSG operation is concluded to prevent other mailbox requests to be performed during that time. If the MSG operation is successfull then the MVI56PDPMV1.Util.MSG.MailboxRequest.DNCounter tag is incremented and the DN bit is cleared. If the MSG is not sucessfull then the MVI56PDPMV1.Util.MSG.MailboxRequest.ERCounter is incremented and the ER bit is cleared. A minimum of 100ms time should be kept between two consecutive requests for better performance, otherwise a MSG error might be returned.
   22: XIC(@1cd415e0@.Command.StartSlaves)XIO(@1cd415e0@.Util.MSG.MailboxRequest.Pending)[[ADD(1,@1cd415e0@.Util.MailboxIDOutLowByte,@1cd415e0@.Util.MailboxIDOutLowByte) ,GEQ(@1cd415e0@.Util.MailboxIDOutLowByte,256) MOV(1,@1cd415e0@.Util.MailboxIDOutLowByte) ,ADD(@1cd415e0@.Util.MailboxIDOutLowByte,-20480,@1cd415e0@.Util.MailboxIDOut) ] ,MOV(@1cd415e0@.Util.MailboxIDOut,@1cd415e0@.Util.MailboxOutBuffer[0]) ,MOV(16386,@1cd415e0@.Util.MailboxOutBuffer[1]) ,MOV(11,@1cd415e0@.Util.MailboxOutBuffer[2]) ,MOV(126,@1cd415e0@.Util.MailboxOutBuffer[3]) ,MOV(1,@1cd415e0@.Util.MailboxOutBuffer[4]) ,MOV(1,@1cd415e0@.Util.MailboxOutBuffer[5]) ,MOV(0,@1cd415e0@.Util.MailboxOutBuffer[6]) ,MOV(0,@1cd415e0@.Util.MailboxOutBuffer[7]) ,MOV(0,@1cd415e0@.Util.MailboxOutBuffer[8]) ,MOV(0,@1cd415e0@.Util.MailboxOutBuffer[9]) ,MOV(0,@1cd415e0@.Util.MailboxOutBuffer[10]) ,MOV(0,@1cd415e0@.Util.MailboxOutBuffer[11]) ,MOV(0,@1cd415e0@.Util.MailboxOutBuffer[12]) ,MOV(0,@1cd415e0@.Util.MailboxOutBuffer[13]) ,MOV(0,@1cd415e0@.Util.MailboxOutBuffer[14]) ,MOV(0,@1cd415e0@.Util.MailboxOutBuffer[15]) ,COP(@1cd415e0@.Mailbox.StartSlaves.Out.SlaveNumber[0],@1cd415e0@.Util.MailboxOutBuffer[16],126) ,XIO(@323855e6@.EN) [MSG(@323855e6@) ,OTL(@1cd415e0@.Util.MSG.MailboxRequest.Pending) ,OTU(@1cd415e0@.Command.StartSlaves) ] ];
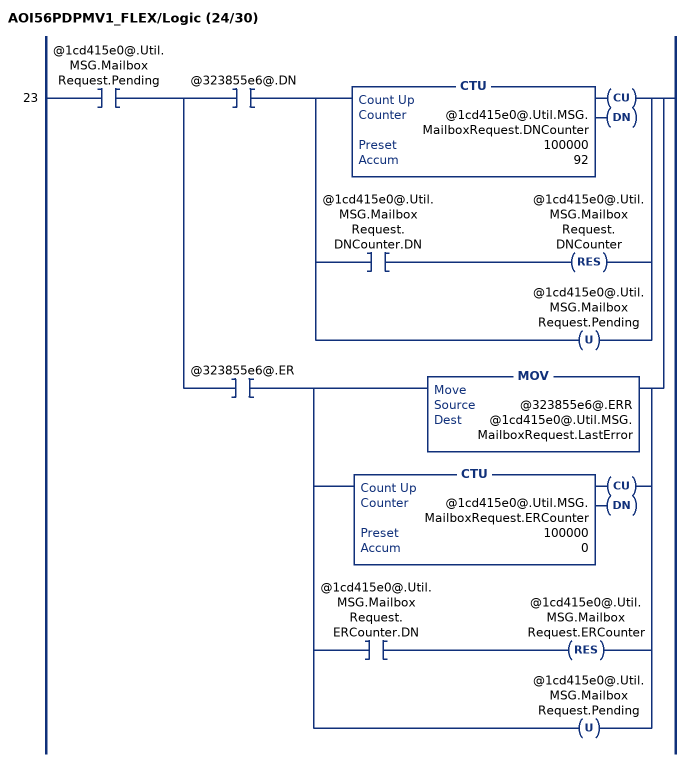
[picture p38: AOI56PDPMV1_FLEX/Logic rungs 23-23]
   23: XIC(@1cd415e0@.Util.MSG.MailboxRequest.Pending)[XIC(@323855e6@.DN) [CTU(@1cd415e0@.Util.MSG.MailboxRequest.DNCounter,100000,92) ,XIC(@1cd415e0@.Util.MSG.MailboxRequest.DNCounter.DN) RES(@1cd415e0@.Util.MSG.MailboxRequest.DNCounter) ,OTU(@1cd415e0@.Util.MSG.MailboxRequest.Pending) ] ,XIC(@323855e6@.ER) [MOV(@323855e6@.ERR,@1cd415e0@.Util.MSG.MailboxRequest.LastError) ,CTU(@1cd415e0@.Util.MSG.MailboxRequest.ERCounter,100000,0) ,XIC(@1cd415e0@.Util.MSG.MailboxRequest.ERCounter.DN) RES(@1cd415e0@.Util.MSG.MailboxRequest.ERCounter) ,OTU(@1cd415e0@.Util.MSG.MailboxRequest.Pending) ] ];
